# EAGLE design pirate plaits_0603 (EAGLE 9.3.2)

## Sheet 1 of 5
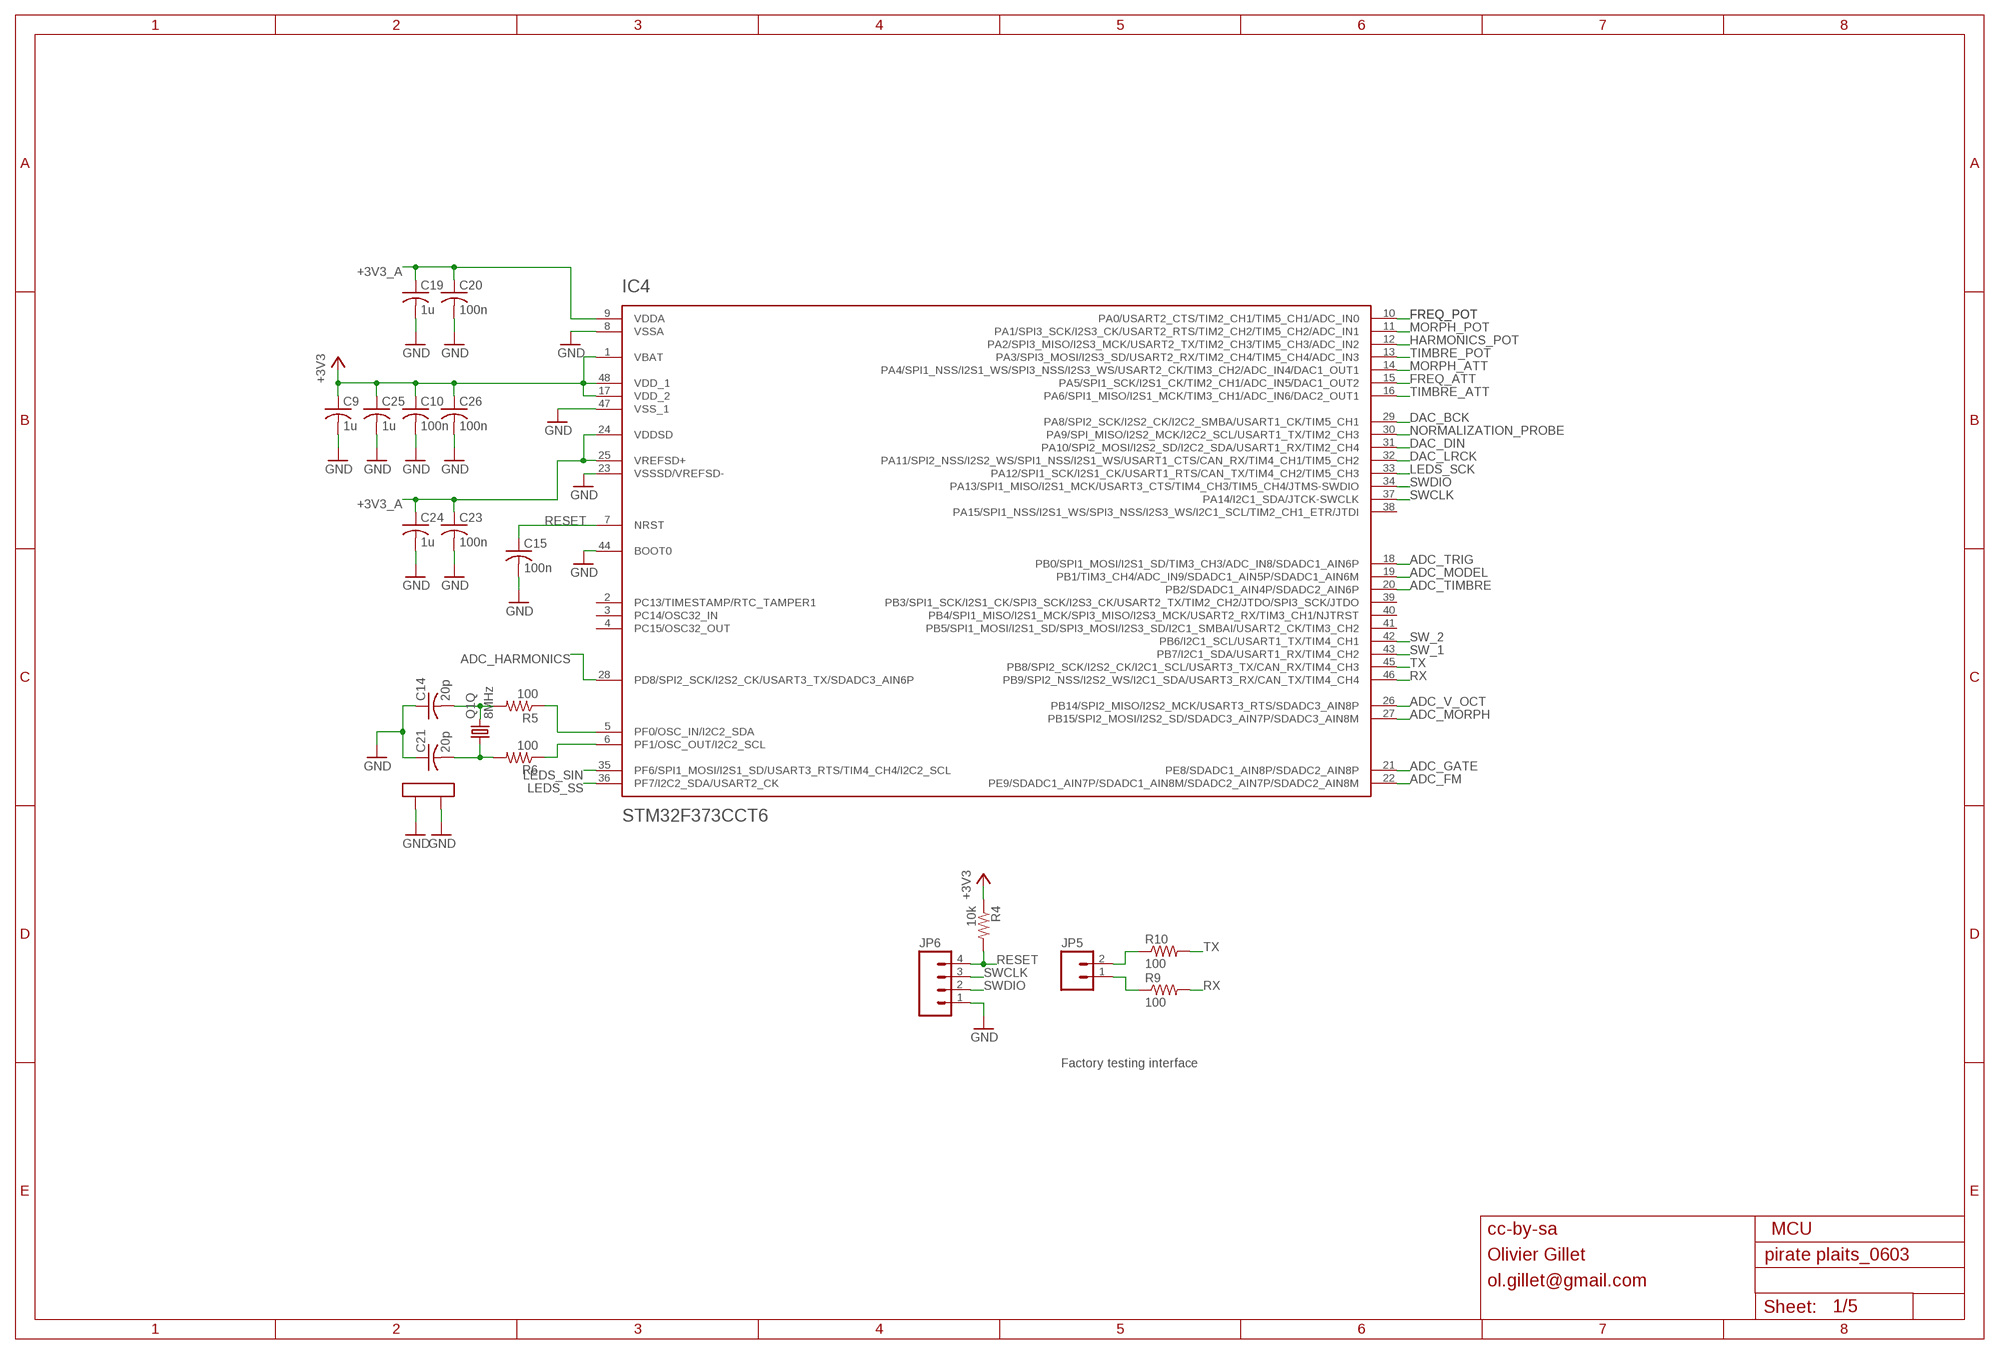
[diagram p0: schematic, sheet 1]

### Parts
C9  1u  C-USC0603  [C0603]
C10  100n  C-USC0603  [C0603]
C14  20p  C-USC0603  [C0603]
C15  100n  C-USC0603  [C0603]
C19  1u  C-USC0603  [C0603]
C20  100n  C-USC0603  [C0603]
C21  20p  C-USC0603  [C0603]
C23  100n  C-USC0603  [C0603]
C24  1u  C-USC0603  [C0603]
C25  1u  C-USC0603  [C0603]
C26  100n  C-USC0603  [C0603]
IC4  STM32F373CCT6  STM32F373C  [LQFP48]
JP5  M02PTH  [1X02]
JP6  M04PTH  [1X04]
Q1  8MHz  CRYSTAL  [CTS406]
R4  10k  R-US_R0603  [R0603]
R5  100  R-US_R0603  [R0603]
R6  100  R-US_R0603  [R0603]
R9  100  R-US_R0603  [R0603]
R10  100  R-US_R0603  [R0603]

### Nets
+3V3: C9.1 C10.1 C25.1 C26.1 IC4.1(VBAT) IC4.17(VDD_2) IC4.48(VDD_1) R4.1 ; also sheet 2,3,4,5
+3V3_A: C19.1 C20.1 C23.1 C24.1 IC4.9(VDDA) IC4.24(VDDSD) IC4.25(VREFSD+) ; also sheet 2,3,4,5
ADC_FM: IC4.22(PE9/SDADC1_AIN7P/SDADC1_AIN8M/SDADC2_AIN7P/SDADC2_AIN8M) ; also sheet 3
ADC_GATE: IC4.21(PE8/SDADC1_AIN8P/SDADC2_AIN8P) ; also sheet 3
ADC_HARMONICS: IC4.28(PD8/SPI2_SCK/I2S2_CK/USART3_TX/SDADC3_AIN6P) ; also sheet 3
ADC_MODEL: IC4.19(PB1/TIM3_CH4/ADC_IN9/SDADC1_AIN5P/SDADC1_AIN6M) ; also sheet 3
ADC_MORPH: IC4.27(PB15/SPI2_MOSI/I2S2_SD/SDADC3_AIN7P/SDADC3_AIN8M) ; also sheet 3
ADC_TIMBRE: IC4.20(PB2/SDADC1_AIN4P/SDADC2_AIN6P) ; also sheet 3
ADC_TRIG: IC4.18(PB0/SPI1_MOSI/I2S1_SD/TIM3_CH3/ADC_IN8/SDADC1_AIN6P) ; also sheet 3
ADC_V_OCT: IC4.26(PB14/SPI2_MISO/I2S2_MCK/USART3_RTS/SDADC3_AIN8P) ; also sheet 3
DAC_BCK: IC4.29(PA8/SPI2_SCK/I2S2_CK/I2C2_SMBA/USART1_CK/TIM5_CH1) ; also sheet 4
DAC_DIN: IC4.31(PA10/SPI2_MOSI/I2S2_SD/I2C2_SDA/USART1_RX/TIM2_CH4) ; also sheet 4
DAC_LRCK: IC4.32(PA11/SPI2_NSS/I2S2_WS/SPI1_NSS/I2S1_WS/USART1_CTS/CAN_RX/TIM4_CH1/TIM5_CH2) ; also sheet 4
FREQ_ATT: IC4.15(PA5/SPI1_SCK/I2S1_CK/TIM2_CH1/ADC_IN5/DAC1_OUT2) ; also sheet 2
FREQ_POT: IC4.10(PA0/USART2_CTS/TIM2_CH1/TIM5_CH1/ADC_IN0) ; also sheet 2
GND: C9.2 C10.2 C14.1 C15.2 C19.2 C20.2 C21.1 C23.2 C24.2 C25.2 C26.2 IC4.8(VSSA) IC4.23(VSSSD/VREFSD-) IC4.44(BOOT0) IC4.47(VSS_1) JP6.1 Q1.2(LID1) Q1.4(LID2) ; also sheet 2,3,4,5
HARMONICS_POT: IC4.12(PA2/SPI3_MISO/I2S3_MCK/USART2_TX/TIM2_CH3/TIM5_CH3/ADC_IN2) ; also sheet 2
LEDS_SCK: IC4.33(PA12/SPI1_SCK/I2S1_CK/USART1_RTS/CAN_TX/TIM4_CH2/TIM5_CH3) ; also sheet 2
LEDS_SIN: IC4.35(PF6/SPI1_MOSI/I2S1_SD/USART3_RTS/TIM4_CH4/I2C2_SCL) ; also sheet 2
LEDS_SS: IC4.36(PF7/I2C2_SDA/USART2_CK) ; also sheet 2
MORPH_ATT: IC4.14(PA4/SPI1_NSS/I2S1_WS/SPI3_NSS/I2S3_WS/USART2_CK/TIM3_CH2/ADC_IN4/DAC1_OUT1) ; also sheet 2
MORPH_POT: IC4.11(PA1/SPI3_SCK/I2S3_CK/USART2_RTS/TIM2_CH2/TIM5_CH2/ADC_IN1) ; also sheet 2
N$7: IC4.5(PF0/OSC_IN/I2C2_SDA) R5.1
N$8: IC4.6(PF1/OSC_OUT/I2C2_SCL) R6.1
N$29: C14.2 Q1.3 R5.2
N$33: JP5.2 R10.1
N$35: C21.2 Q1.1 R6.2
N$51: JP5.1 R9.1
NORMALIZATION_PROBE: IC4.30(PA9/SPI_MISO/I2S2_MCK/I2C2_SCL/USART1_TX/TIM2_CH3) ; also sheet 3
RESET: C15.1 IC4.7(NRST) JP6.4 R4.2
RX: IC4.46(PB9/SPI2_NSS/I2S2_WS/I2C1_SDA/USART3_RX/CAN_TX/TIM4_CH4) R9.2
SW_1: IC4.43(PB7/I2C1_SDA/USART1_RX/TIM4_CH2) ; also sheet 2
SW_2: IC4.42(PB6/I2C1_SCL/USART1_TX/TIM4_CH1) ; also sheet 2
SWCLK: IC4.37(PA14/I2C1_SDA/JTCK-SWCLK) JP6.3
SWDIO: IC4.34(PA13/SPI1_MISO/I2S1_MCK/USART3_CTS/TIM4_CH3/TIM5_CH4/JTMS-SWDIO) JP6.2
TIMBRE_ATT: IC4.16(PA6/SPI1_MISO/I2S1_MCK/TIM3_CH1/ADC_IN6/DAC2_OUT1) ; also sheet 2
TIMBRE_POT: IC4.13(PA3/SPI3_MOSI/I2S3_SD/USART2_RX/TIM2_CH4/TIM5_CH4/ADC_IN3) ; also sheet 2
TX: IC4.45(PB8/SPI2_SCK/I2S2_CK/I2C1_SCL/USART3_TX/CAN_RX/TIM4_CH3) R10.2
Unconnected: IC4.2(PC13/TIMESTAMP/RTC_TAMPER1) IC4.3(PC14/OSC32_IN) IC4.4(PC15/OSC32_OUT) IC4.38(PA15/SPI1_NSS/I2S1_WS/SPI3_NSS/I2S3_WS/I2C1_SCL/TIM2_CH1_ETR/JTDI) IC4.39(PB3/SPI1_SCK/I2S1_CK/SPI3_SCK/I2S3_CK/USART2_TX/TIM2_CH2/JTDO/SPI3_SCK/JTDO) IC4.40(PB4/SPI1_MISO/I2S1_MCK/SPI3_MISO/I2S3_MCK/USART2_RX/TIM3_CH1/NJTRST) IC4.41(PB5/SPI1_MOSI/I2S1_SD/SPI3_MOSI/I2S3_SD/I2C1_SMBAI/USART2_CK/TIM3_CH2)

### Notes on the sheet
- Factory testing interface
- cc-by-sa | MCU
- Olivier Gillet
- ol.gillet@gmail.com

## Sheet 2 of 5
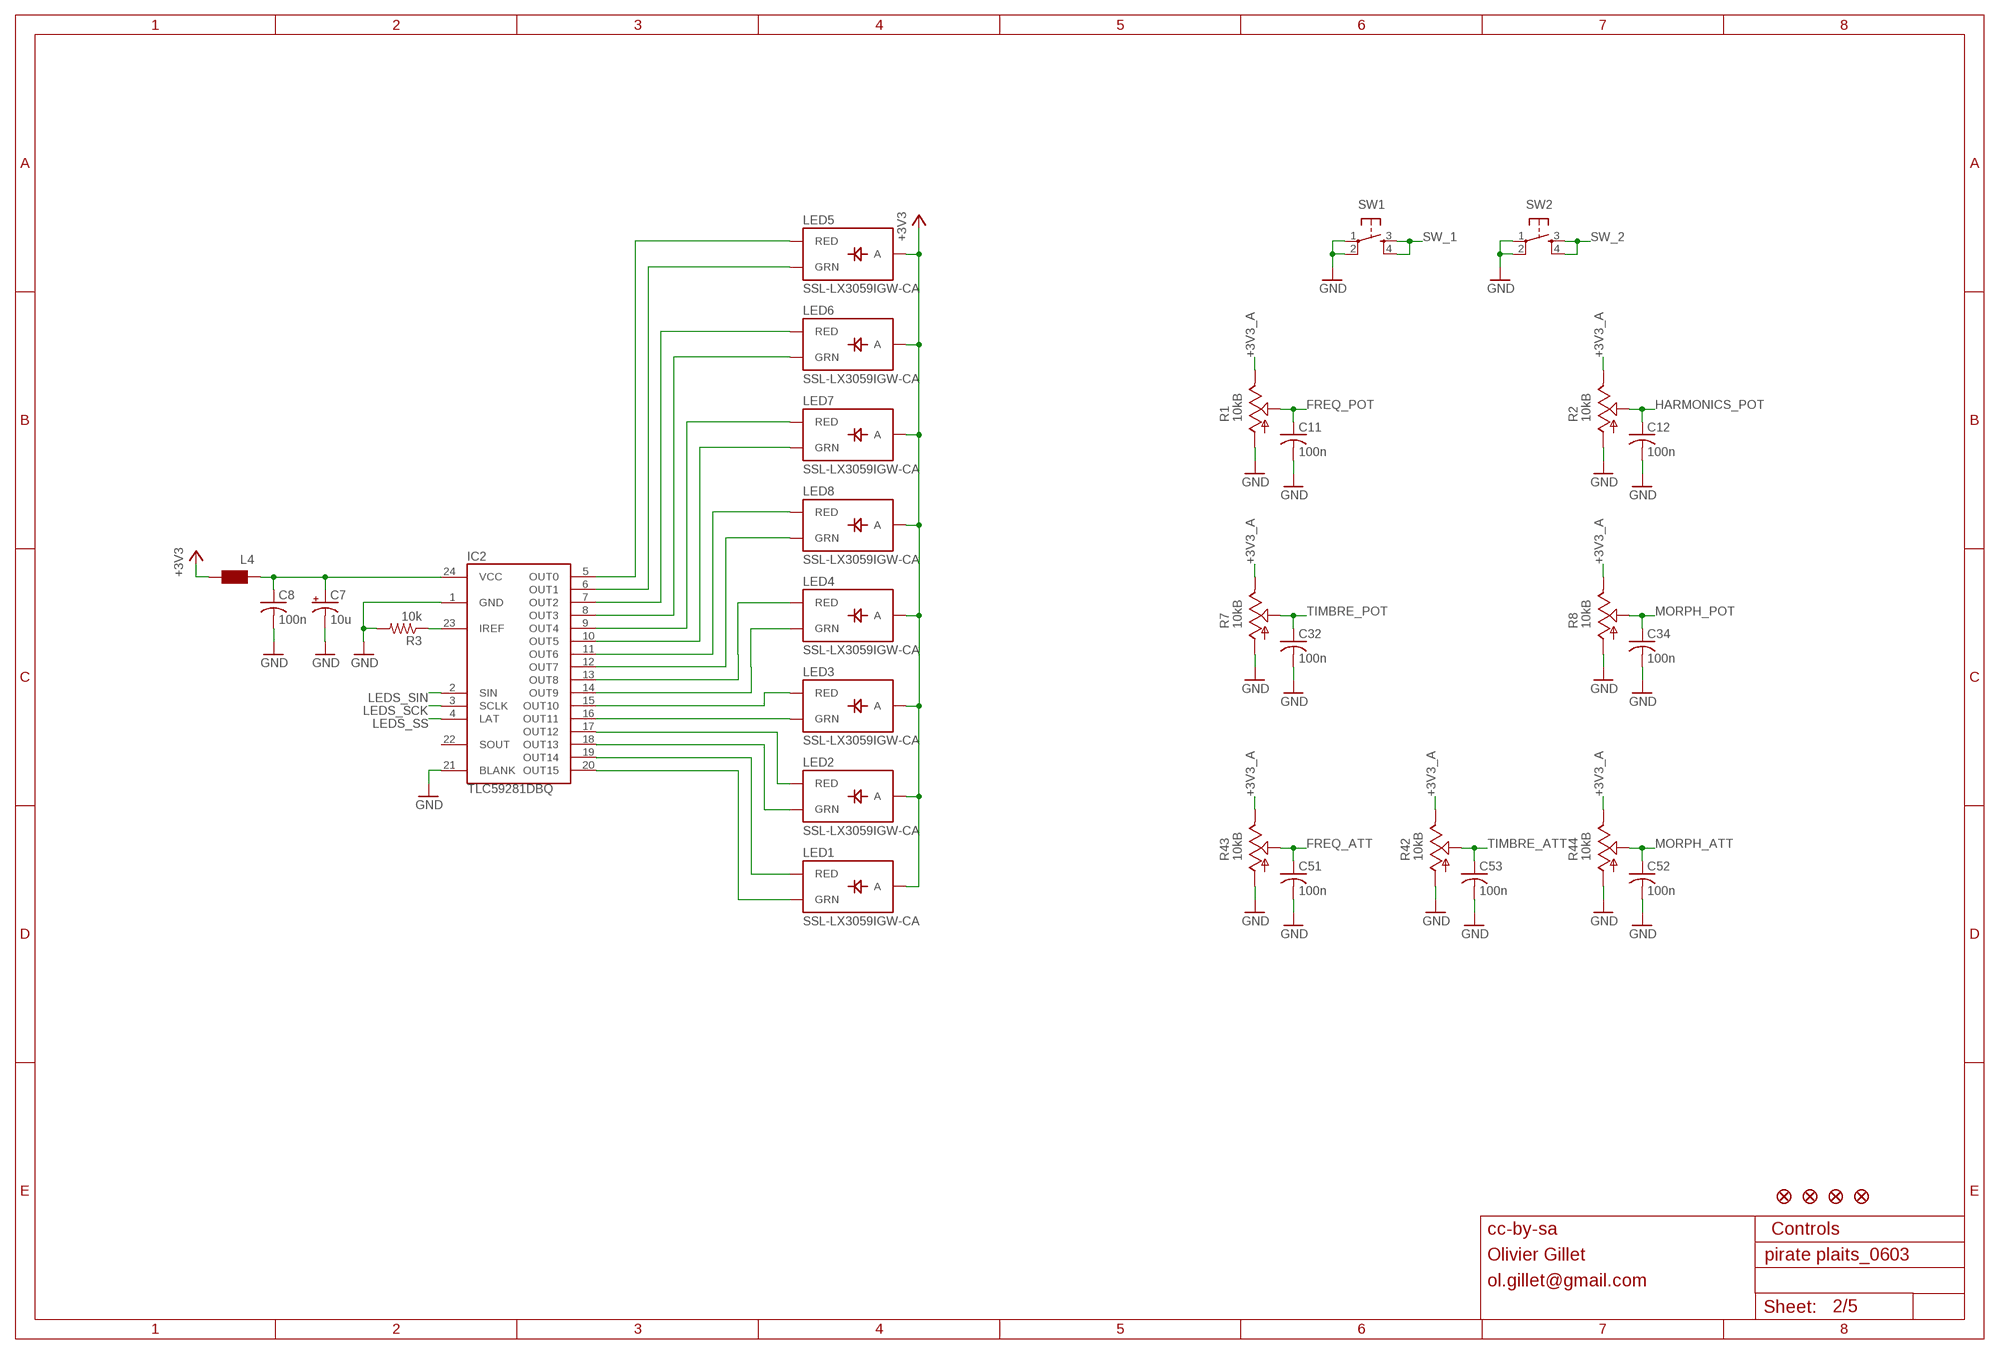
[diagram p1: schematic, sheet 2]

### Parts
C7  10u  CPOL-USA  [PANASONIC_A]
C8  100n  C-USC0603  [C0603]
C11  100n  C-USC0603  [C0603]
C12  100n  C-USC0603  [C0603]
C32  100n  C-USC0603  [C0603]
C34  100n  C-USC0603  [C0603]
C51  100n  C-USC0603  [C0603]
C52  100n  C-USC0603  [C0603]
C53  100n  C-USC0603  [C0603]
IC2  TLC59281DBQ  [TSSOP24_0635]
JP1  FIDUCIAL1X2  [FIDUCIAL-1X2]
JP2  FIDUCIAL1X2  [FIDUCIAL-1X2]
JP3  FIDUCIAL1X2  [FIDUCIAL-1X2]
JP4  FIDUCIAL1X2  [FIDUCIAL-1X2]
L4  WE-CBF_0603  [0603]
LED1  SSL-LX3059IGW-CA  LED-BICOLOR-THROUGHHOLE-CA  [LED-BICOLOR-THROUGHHOLE-LUMEX]
LED2  SSL-LX3059IGW-CA  LED-BICOLOR-THROUGHHOLE-CA  [LED-BICOLOR-THROUGHHOLE-LUMEX]
LED3  SSL-LX3059IGW-CA  LED-BICOLOR-THROUGHHOLE-CA  [LED-BICOLOR-THROUGHHOLE-LUMEX]
LED4  SSL-LX3059IGW-CA  LED-BICOLOR-THROUGHHOLE-CA  [LED-BICOLOR-THROUGHHOLE-LUMEX]
LED5  SSL-LX3059IGW-CA  LED-BICOLOR-THROUGHHOLE-CA  [LED-BICOLOR-THROUGHHOLE-LUMEX]
LED6  SSL-LX3059IGW-CA  LED-BICOLOR-THROUGHHOLE-CA  [LED-BICOLOR-THROUGHHOLE-LUMEX]
LED7  SSL-LX3059IGW-CA  LED-BICOLOR-THROUGHHOLE-CA  [LED-BICOLOR-THROUGHHOLE-LUMEX]
LED8  SSL-LX3059IGW-CA  LED-BICOLOR-THROUGHHOLE-CA  [LED-BICOLOR-THROUGHHOLE-LUMEX]
R1  10kB  POT_USVERTICAL_PS  [ALPS_POT_VERTICAL_PS]
R2  10kB  POT_USVERTICAL_PS  [ALPS_POT_VERTICAL_PS]
R3  10k  R-US_R0603  [R0603]
R7  10kB  POT_USVERTICAL_PS  [ALPS_POT_VERTICAL_PS]
R8  10kB  POT_USVERTICAL_PS  [ALPS_POT_VERTICAL_PS]
R42  10kB  POT_USVERTICAL  [ALPS_POT_VERTICAL]
R43  10kB  POT_USVERTICAL  [ALPS_POT_VERTICAL]
R44  10kB  POT_USVERTICAL  [ALPS_POT_VERTICAL]
SW1  TAC_SWITCHPTH  [TACTILE-PTH]
SW2  TAC_SWITCHPTH  [TACTILE-PTH]

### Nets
+3V3: L4.2 LED1.A LED2.A LED3.A LED4.A LED5.A LED6.A LED7.A LED8.A ; also sheet 1,3,4,5
+3V3_A: R1.P$1(E) R2.P$1(E) R7.P$1(E) R8.P$1(E) R42.P$1(E) R43.P$1(E) R44.P$1(E) ; also sheet 1,3,4,5
FREQ_ATT: C51.1 R43.P$2(S) ; also sheet 1
FREQ_POT: C11.1 R1.P$2(S) ; also sheet 1
GND: C7.- C8.2 C11.2 C12.2 C32.2 C34.2 C51.2 C52.2 C53.2 IC2.1(GND) IC2.21(BLANK) R1.P$3(A) R2.P$3(A) R3.2 R7.P$3(A) R8.P$3(A) R42.P$3(A) R43.P$3(A) R44.P$3(A) SW1.1 SW1.2 SW2.1 SW2.2 ; also sheet 1,3,4,5
HARMONICS_POT: C12.1 R2.P$2(S) ; also sheet 1
LEDS_SCK: IC2.3(SCLK) ; also sheet 1
LEDS_SIN: IC2.2(SIN) ; also sheet 1
LEDS_SS: IC2.4(LAT) ; also sheet 1
MORPH_ATT: C52.1 R44.P$2(S) ; also sheet 1
MORPH_POT: C34.1 R8.P$2(S) ; also sheet 1
N$2: IC2.12(OUT7) LED8.GREEN_C(GRN)
N$5: IC2.11(OUT6) LED8.RED_C(RED)
N$9: IC2.10(OUT5) LED7.GREEN_C(GRN)
N$10: IC2.9(OUT4) LED7.RED_C(RED)
N$11: IC2.8(OUT3) LED6.GREEN_C(GRN)
N$12: IC2.13(OUT8) LED4.RED_C(RED)
N$13: IC2.7(OUT2) LED6.RED_C(RED)
N$14: IC2.14(OUT9) LED4.GREEN_C(GRN)
N$15: IC2.6(OUT1) LED5.GREEN_C(GRN)
N$17: IC2.15(OUT10) LED3.RED_C(RED)
N$18: IC2.16(OUT11) LED3.GREEN_C(GRN)
N$19: IC2.17(OUT12) LED2.RED_C(RED)
N$20: IC2.18(OUT13) LED2.GREEN_C(GRN)
N$21: IC2.19(OUT14) LED1.RED_C(RED)
N$22: IC2.5(OUT0) LED5.RED_C(RED)
N$23: IC2.20(OUT15) LED1.GREEN_C(GRN)
N$27: C7.+ C8.1 IC2.24(VCC) L4.1
N$68: IC2.23(IREF) R3.1
SW_1: SW1.3 SW1.4 ; also sheet 1
SW_2: SW2.3 SW2.4 ; also sheet 1
TIMBRE_ATT: C53.1 R42.P$2(S) ; also sheet 1
TIMBRE_POT: C32.1 R7.P$2(S) ; also sheet 1
Unconnected: IC2.22(SOUT)

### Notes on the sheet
- cc-by-sa | Controls
- Olivier Gillet
- ol.gillet@gmail.com

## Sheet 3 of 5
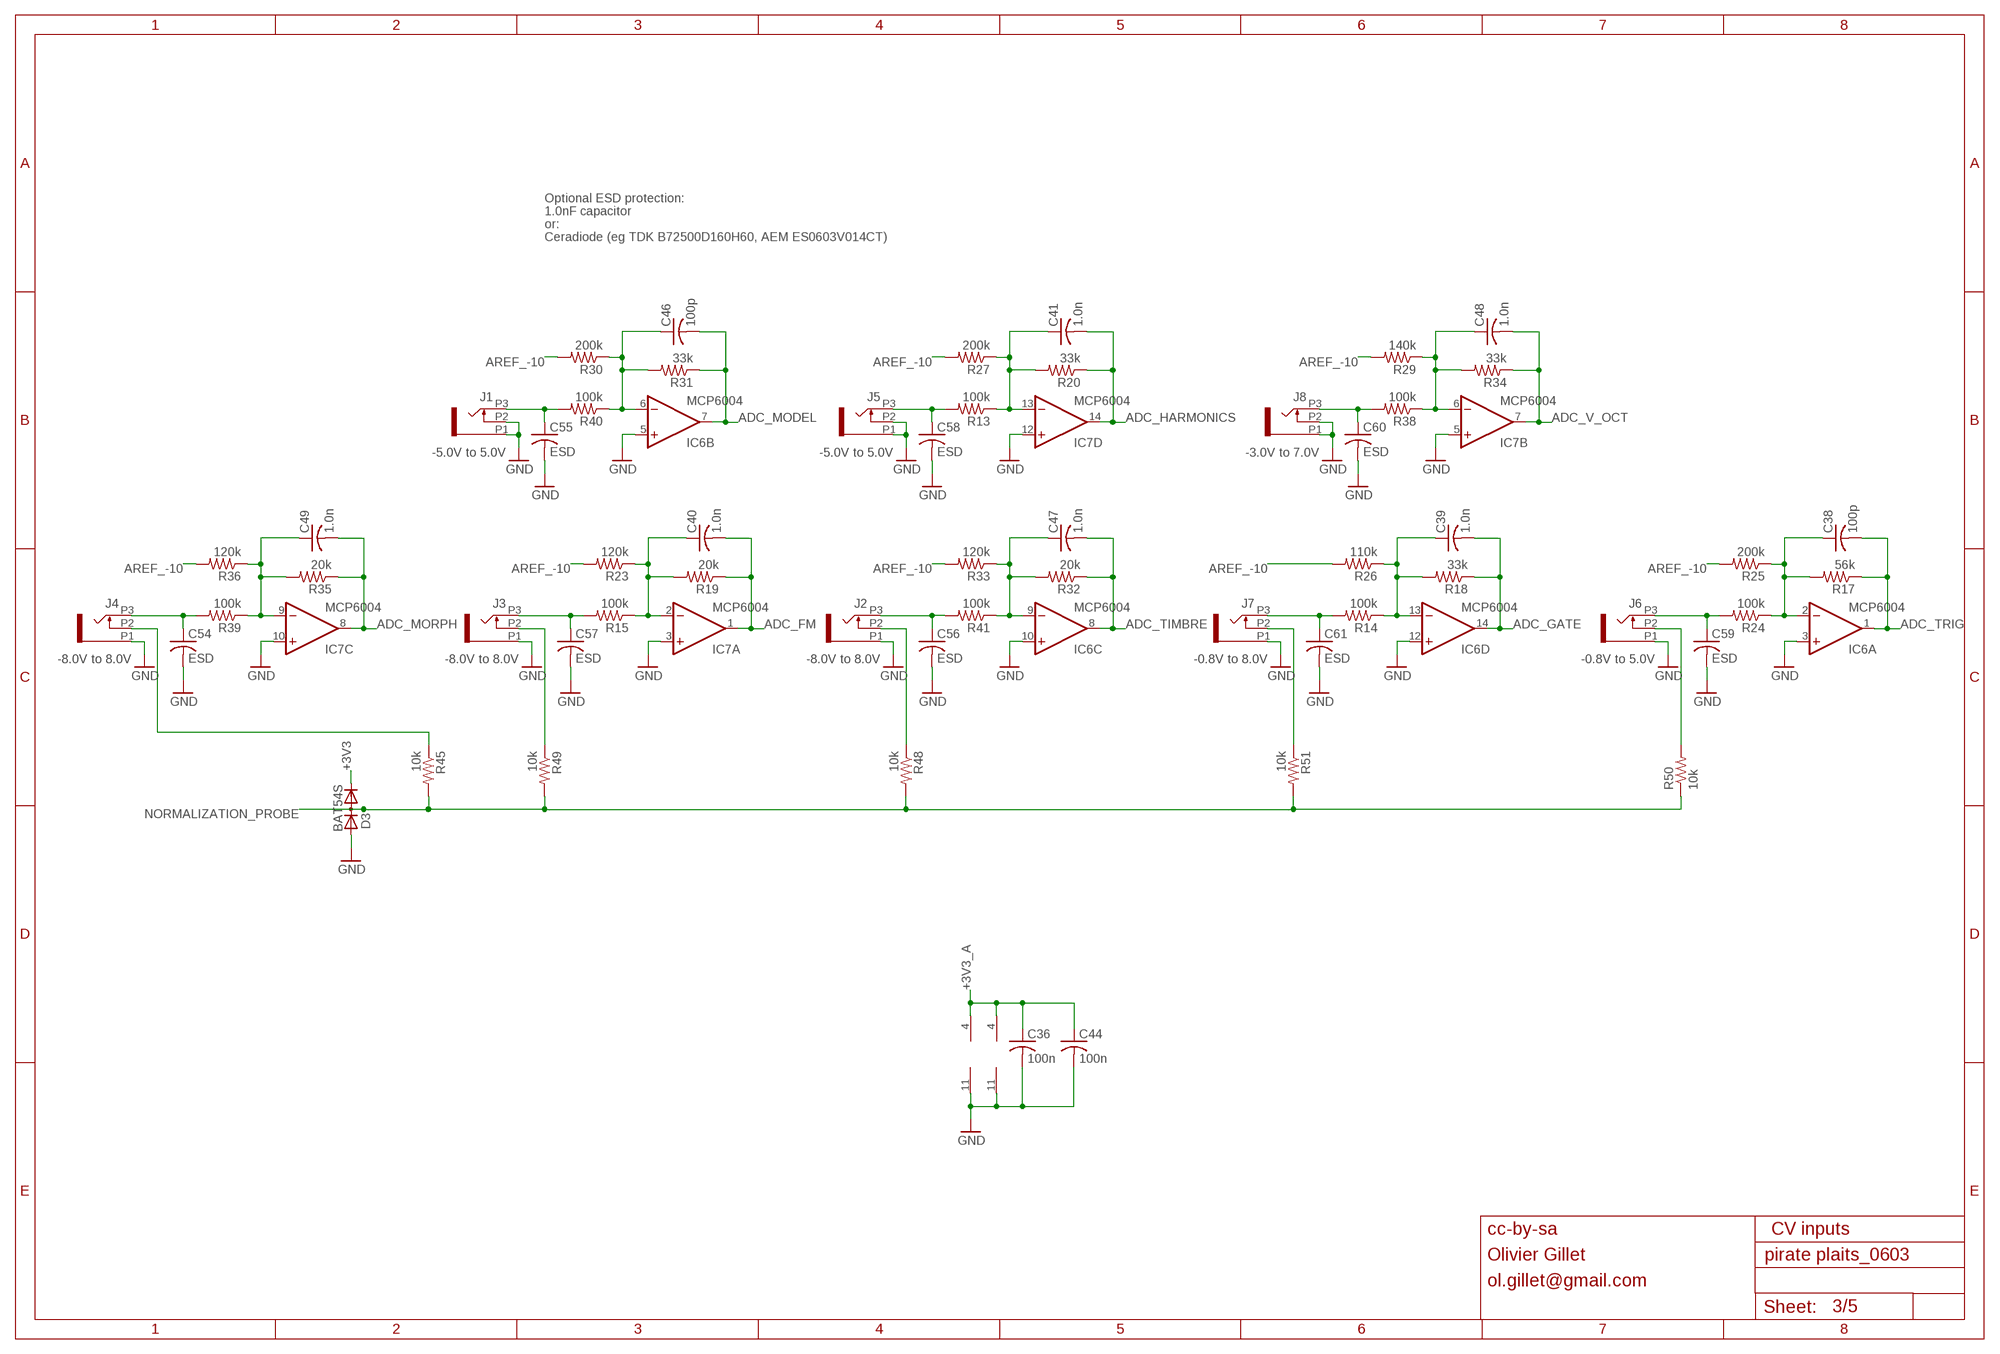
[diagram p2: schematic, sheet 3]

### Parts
C36  100n  C-USC0603  [C0603]
C38  100p  C-USC0603  [C0603]
C39  1.0n  C-USC0603  [C0603]
C40  1.0n  C-USC0603  [C0603]
C41  1.0n  C-USC0603  [C0603]
C44  100n  C-USC0603  [C0603]
C46  100p  C-USC0603  [C0603]
C47  1.0n  C-USC0603  [C0603]
C48  1.0n  C-USC0603  [C0603]
C49  1.0n  C-USC0603  [C0603]
C54  ESD  C-USC0603  [C0603]
C55  ESD  C-USC0603  [C0603]
C56  ESD  C-USC0603  [C0603]
C57  ESD  C-USC0603  [C0603]
C58  ESD  C-USC0603  [C0603]
C59  ESD  C-USC0603  [C0603]
C60  ESD  C-USC0603  [C0603]
C61  ESD  C-USC0603  [C0603]
D3  BAT54S  DIODE_2CACA-SOT23  [SOT23]
IC6  MCP6004  TL074PW  [TSSOP14_065]
IC7  MCP6004  TL074PW  [TSSOP14_065]
J1  PJ301_THONKICONN6  [WQP_PJ_301M6]
J2  PJ301_THONKICONN6  [WQP_PJ_301M6]
J3  PJ301_THONKICONN6  [WQP_PJ_301M6]
J4  PJ301_THONKICONN6  [WQP_PJ_301M6]
J5  PJ301_THONKICONN6  [WQP_PJ_301M6]
J6  PJ301_THONKICONN6  [WQP_PJ_301M6]
J7  PJ301_THONKICONN6  [WQP_PJ_301M6]
J8  PJ301_THONKICONN6  [WQP_PJ_301M6]
R13  100k  R-US_R0603  [R0603]
R14  100k  R-US_R0603  [R0603]
R15  100k  R-US_R0603  [R0603]
R17  56k  R-US_R0603  [R0603]
R18  33k  R-US_R0603  [R0603]
R19  20k  R-US_R0603  [R0603]
R20  33k  R-US_R0603  [R0603]
R23  120k  R-US_R0603  [R0603]
R24  100k  R-US_R0603  [R0603]
R25  200k  R-US_R0603  [R0603]
R26  110k  R-US_R0603  [R0603]
R27  200k  R-US_R0603  [R0603]
R29  140k  R-US_R0603  [R0603]
R30  200k  R-US_R0603  [R0603]
R31  33k  R-US_R0603  [R0603]
R32  20k  R-US_R0603  [R0603]
R33  120k  R-US_R0603  [R0603]
R34  33k  R-US_R0603  [R0603]
R35  20k  R-US_R0603  [R0603]
R36  120k  R-US_R0603  [R0603]
R38  100k  R-US_R0603  [R0603]
R39  100k  R-US_R0603  [R0603]
R40  100k  R-US_R0603  [R0603]
R41  100k  R-US_R0603  [R0603]
R45  10k  R-US_R0603  [R0603]
R48  10k  R-US_R0603  [R0603]
R49  10k  R-US_R0603  [R0603]
R50  10k  R-US_R0603  [R0603]
R51  10k  R-US_R0603  [R0603]

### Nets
+3V3: D3.2(C) ; also sheet 1,2,4,5
+3V3_A: C36.1 C44.1 IC6.4(P:V+) IC7.4(P:V+) ; also sheet 1,2,4,5
ADC_FM: C40.2 IC7.1(A:OUT) R19.1 ; also sheet 1
ADC_GATE: C39.2 IC6.14(D:OUT) R18.1 ; also sheet 1
ADC_HARMONICS: C41.2 IC7.14(D:OUT) R20.1 ; also sheet 1
ADC_MODEL: C46.2 IC6.7(B:OUT) R31.1 ; also sheet 1
ADC_MORPH: C49.2 IC7.8(C:OUT) R35.1 ; also sheet 1
ADC_TIMBRE: C47.2 IC6.8(C:OUT) R32.1 ; also sheet 1
ADC_TRIG: C38.2 IC6.1(A:OUT) R17.1 ; also sheet 1
ADC_V_OCT: C48.2 IC7.7(B:OUT) R34.1 ; also sheet 1
AREF_-10: R23.2 R25.2 R26.2 R27.2 R29.2 R30.2 R33.2 R36.2 ; also sheet 5
FM_IN: C57.1 J3.P3 R15.2
GATE_IN: C61.1 J7.P3 R14.2
GATE_IN1: C59.1 J6.P3 R24.2
GND: C36.2 C44.2 C54.2 C55.2 C56.2 C57.2 C58.2 C59.2 C60.2 C61.2 D3.1(A) IC6.3(A:+IN) IC6.5(B:+IN) IC6.10(C:+IN) IC6.11(P:V-) IC6.12(D:+IN) IC7.3(A:+IN) IC7.5(B:+IN) IC7.10(C:+IN) IC7.11(P:V-) IC7.12(D:+IN) J1.P1 J1.P2 J2.P1 J3.P1 J4.P1 J5.P1 J5.P2 J6.P1 J7.P1 J8.P1 J8.P2 ; also sheet 1,2,4,5
HARMONICS_IN: C58.1 J5.P3 R13.2
MODEL_IN: C55.1 J1.P3 R40.2
MORPH_IN: C54.1 J4.P3 R39.2
N$3: J6.P2 R50.2
N$4: C38.1 IC6.2(A:-IN) R17.2 R24.1 R25.1
N$24: J3.P2 R49.1
N$25: J2.P2 R48.1
N$26: J4.P2 R45.1
N$28: C39.1 IC6.13(D:-IN) R14.1 R18.2 R26.1
N$30: C48.1 IC7.6(B:-IN) R29.1 R34.2 R38.1
N$31: C56.1 J2.P3 R41.2
N$32: C49.1 IC7.9(C:-IN) R35.2 R36.1 R39.1
N$34: C40.1 IC7.2(A:-IN) R15.1 R19.2 R23.1
N$36: J7.P2 R51.1
N$37: C46.1 IC6.6(B:-IN) R30.1 R31.2 R40.1
N$39: C47.1 IC6.9(C:-IN) R32.2 R33.1 R41.1
N$41: C41.1 IC7.13(D:-IN) R13.1 R20.2 R27.1
NORMALIZATION_PROBE: D3.3(AC) R45.2 R48.2 R49.2 R50.1 R51.2 ; also sheet 1
V_OCT_IN: C60.1 J8.P3 R38.2

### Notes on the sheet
- Optional ESD protection:
- 1.0nF capacitor
- or:
- Ceradiode (eg TDK B72500D160H60, AEM ES0603V014CT)
- -5.0V to 5.0V | -5.0V to 5.0V | -3.0V to 7.0V
- -8.0V to 8.0V | -8.0V to 8.0V | -8.0V to 8.0V | -0.8V to 8.0V | -0.8V to 5.0V
- cc-by-sa | CV inputs
- Olivier Gillet
- ol.gillet@gmail.com

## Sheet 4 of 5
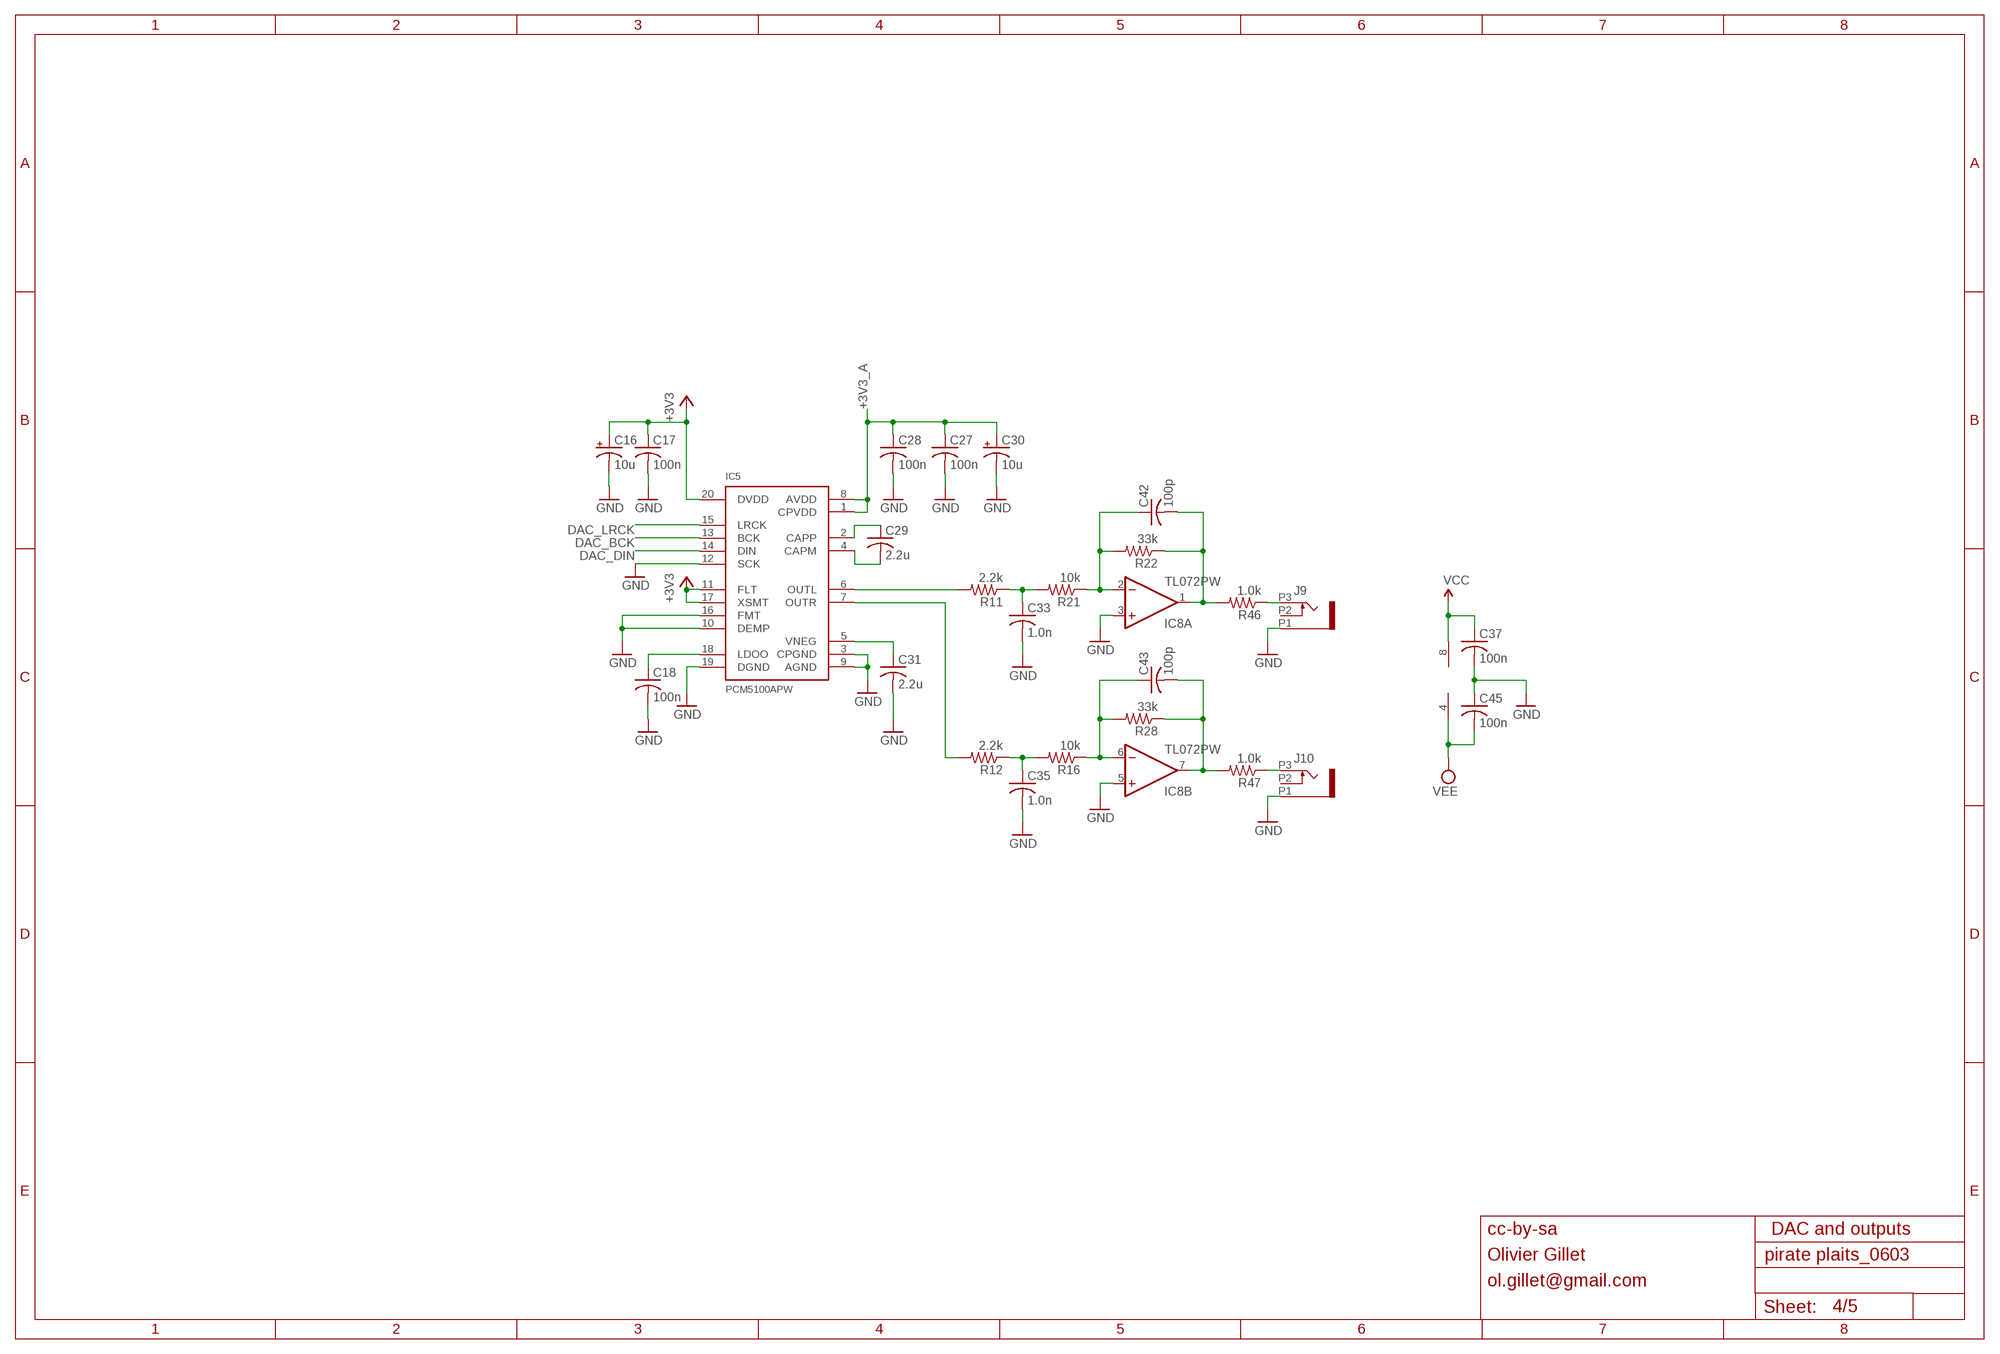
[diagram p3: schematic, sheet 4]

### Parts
C16  10u  CPOL-USA  [PANASONIC_A]
C17  100n  C-USC0603  [C0603]
C18  100n  C-USC0603  [C0603]
C27  100n  C-USC0603  [C0603]
C28  100n  C-USC0603  [C0603]
C29  2.2u  C-USC0805  [C0805]
C30  10u  CPOL-USA  [PANASONIC_A]
C31  2.2u  C-USC0805  [C0805]
C33  1.0n  C-USC0603  [C0603]
C35  1.0n  C-USC0603  [C0603]
C37  100n  C-USC0603  [C0603]
C42  100p  C-USC0603  [C0603]
C43  100p  C-USC0603  [C0603]
C45  100n  C-USC0603  [C0603]
IC5  PCM5100APW  PCM5100PW  [SSOP20]
IC8  TL072PW  [TSSOP08]
J9  PJ301_THONKICONN6  [WQP_PJ_301M6]
J10  PJ301_THONKICONN6  [WQP_PJ_301M6]
R11  2.2k  R-US_R0603  [R0603]
R12  2.2k  R-US_R0603  [R0603]
R16  10k  R-US_R0603  [R0603]
R21  10k  R-US_R0603  [R0603]
R22  33k  R-US_R0603  [R0603]
R28  33k  R-US_R0603  [R0603]
R46  1.0k  R-US_R0603  [R0603]
R47  1.0k  R-US_R0603  [R0603]

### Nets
+3V3: C16.+ C17.1 IC5.11(FLT) IC5.17(XSMT) IC5.20(DVDD) ; also sheet 1,2,3,5
+3V3_A: C27.1 C28.1 C30.+ IC5.1(CPVDD) IC5.8(AVDD) ; also sheet 1,2,3,5
DAC_BCK: IC5.13(BCK) ; also sheet 1
DAC_DIN: IC5.14(DIN) ; also sheet 1
DAC_LRCK: IC5.15(LRCK) ; also sheet 1
GND: C16.- C17.2 C18.2 C27.2 C28.2 C30.- C31.2 C33.2 C35.2 C37.2 C45.1 IC5.3(CPGND) IC5.9(AGND) IC5.10(DEMP) IC5.12(SCK) IC5.16(FMT) IC5.19(DGND) IC8.3(A:+IN) IC8.5(B:+IN) J9.P1 J10.P1 ; also sheet 1,2,3,5
N$6: C29.1 IC5.2(CAPP)
N$16: C29.2 IC5.4(CAPM)
N$43: IC5.6(OUTL) R11.2
N$46: C33.1 R11.1 R21.2
N$47: C35.1 R12.1 R16.2
N$48: C31.1 IC5.5(VNEG)
N$54: C18.1 IC5.18(LDOO)
N$55: IC5.7(OUTR) R12.2
N$58: C43.1 IC8.6(B:-IN) R16.1 R28.2
N$60: C43.2 IC8.7(B:OUT) R28.1 R47.2
N$62: C42.1 IC8.2(A:-IN) R21.1 R22.2
N$63: C42.2 IC8.1(A:OUT) R22.1 R46.2
N$65: J9.P3 R46.1
N$69: J10.P3 R47.1
VCC: C37.1 IC8.8(P:V+) ; also sheet 5
VEE: C45.2 IC8.4(P:V-) ; also sheet 5
Unconnected: J9.P2 J10.P2

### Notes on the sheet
- cc-by-sa | DAC and outputs
- Olivier Gillet
- ol.gillet@gmail.com

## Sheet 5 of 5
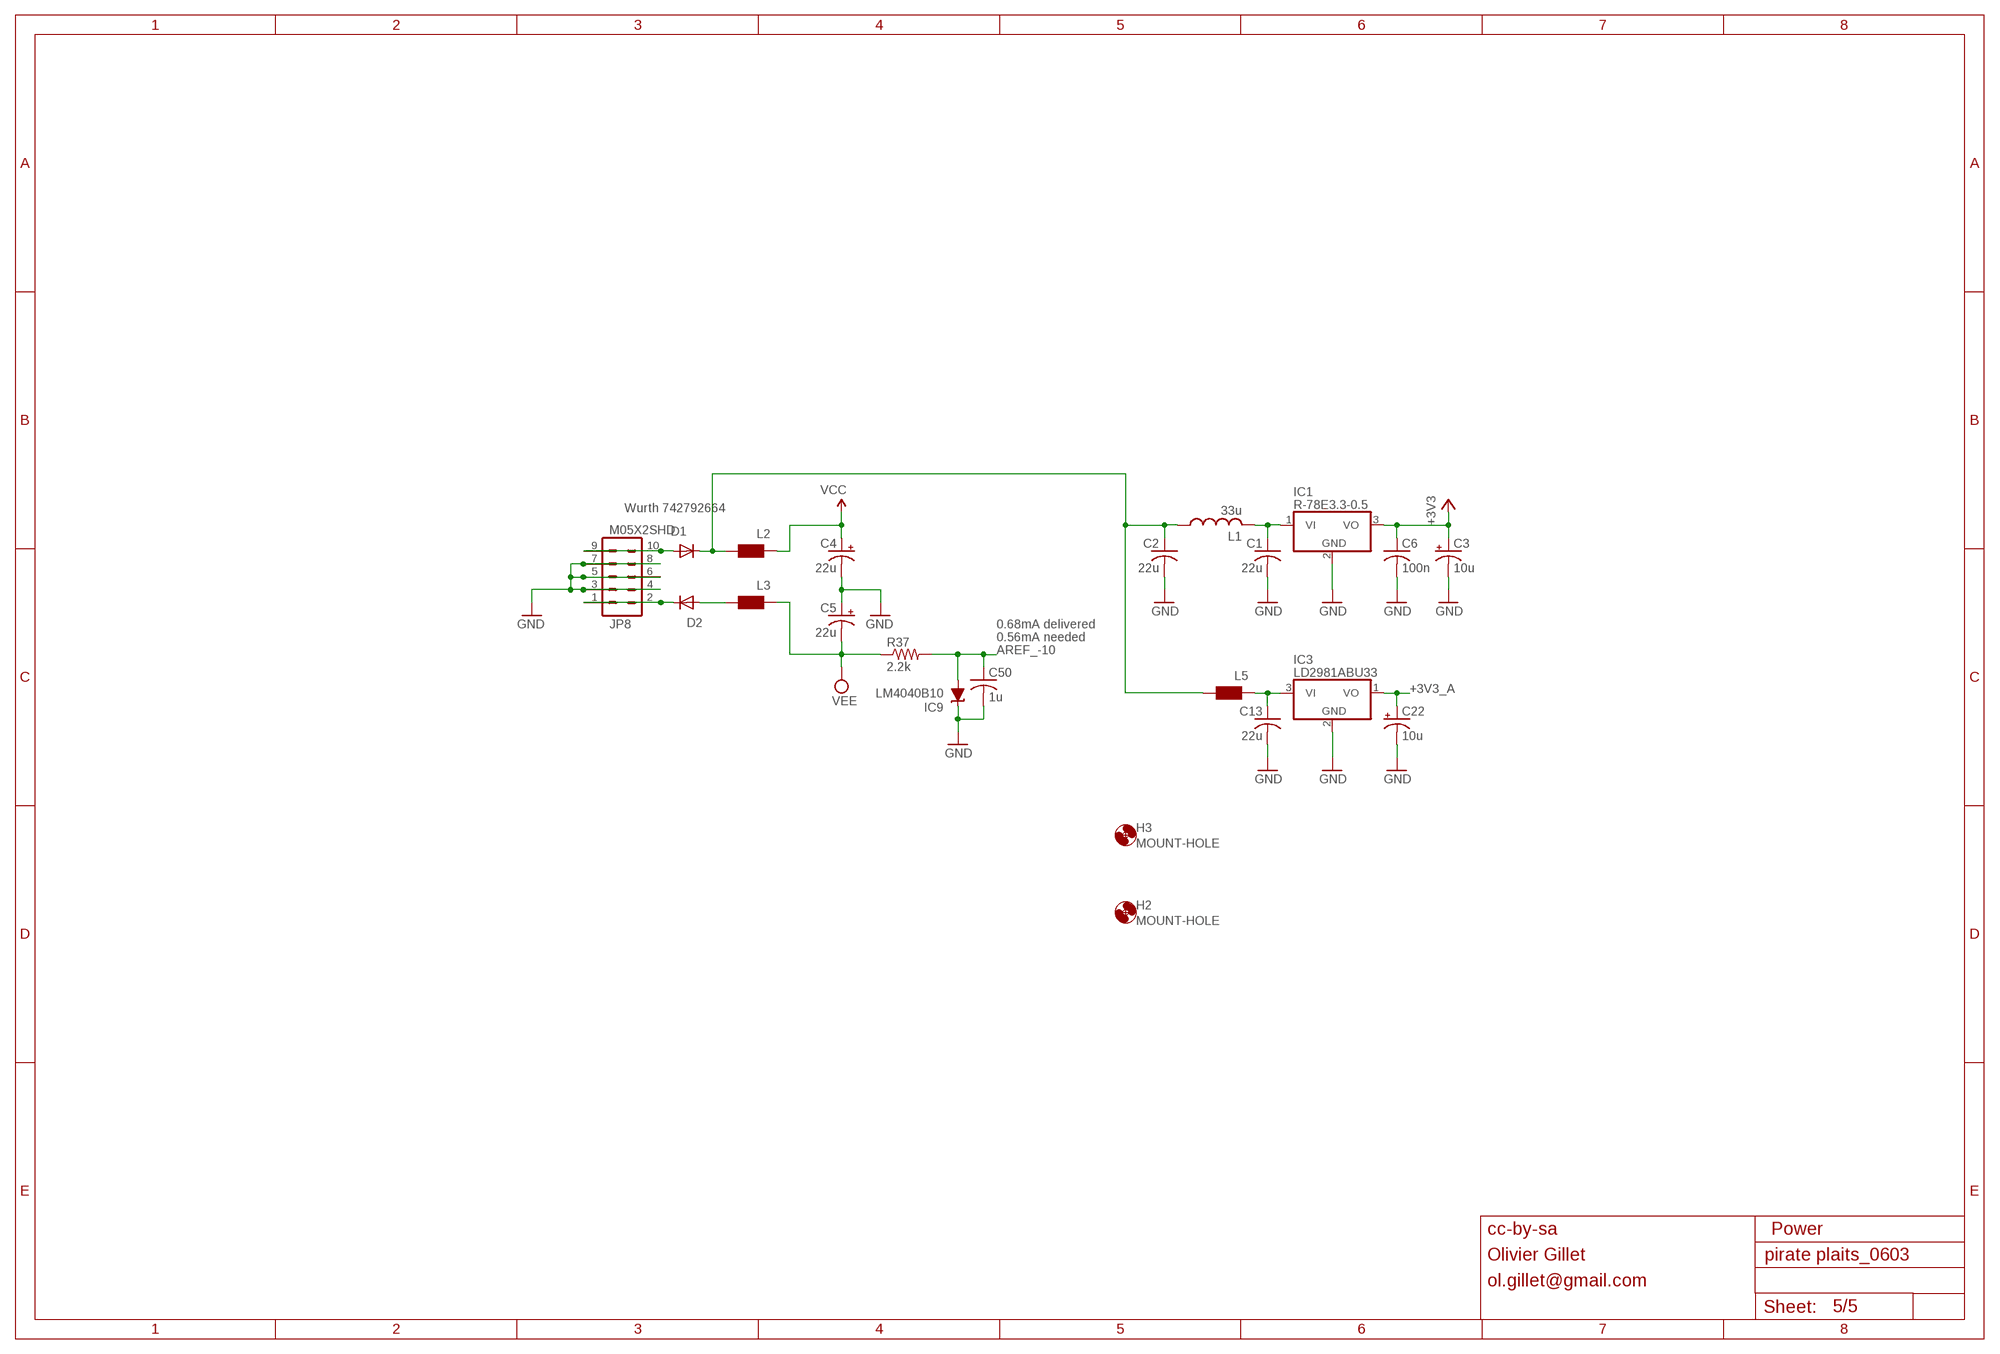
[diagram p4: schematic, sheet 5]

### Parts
C1  22u  C-USC1206  [C1206]
C2  22u  C-USC1206  [C1206]
C3  10u  CPOL-USA  [PANASONIC_A]
C4  22u  CPOL-USB  [PANASONIC_B]
C5  22u  CPOL-USB  [PANASONIC_B]
C6  100n  C-USC0603  [C0603]
C13  22u  C-USC1206  [C1206]
C22  10u  CPOL-USA  [PANASONIC_A]
C50  1u  C-USC0603  [C0603]
D1  1N5819HW  DIODE-SOD123  [SOD123]
D2  1N5819HW  DIODE-SOD123  [SOD123]
H2  MOUNT-HOLE  MOUNT-HOLE3.0TINY  [3,0TINY]
H3  MOUNT-HOLE  MOUNT-HOLE3.0TINY  [3,0TINY]
IC1  R-78E3.3-0.5  WE173950378  [WE78]
IC3  LD2981ABU33  LD2981ABU  [SOT89]
IC9  LM4040B10  LM4041B12DBZ  [DBZ_R-PDSO-G3]
JP8  M05X2SHD  [2X5-SHROUDED]
L1  33u  L-USL2012C  [L2012C]
L2  WE-CBF_0603  [0603]
L3  WE-CBF_0603  [0603]
L5  WE-CBF_0603  [0603]
R37  2.2k  R-US_R0603  [R0603]

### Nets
+3V3: C3.+ C6.1 IC1.3(VO) ; also sheet 1,2,3,4
+3V3_A: C22.+ IC3.1(VO) ; also sheet 1,2,3,4
AREF_-10: C50.1 IC9.2(A) R37.2 ; also sheet 3
GND: C1.2 C2.2 C3.- C4.- C5.+ C6.2 C13.2 C22.- C50.2 IC1.2(GND) IC3.2(GND) IC9.1(C) JP8.3 JP8.4 JP8.5 JP8.6 JP8.7 JP8.8 ; also sheet 1,2,3,4
N$1: C1.1 IC1.1(VI) L1.2
N$38: D2.A L3.2
N$40: C2.1 D1.C L1.1 L2.2 L5.2
N$42: C13.1 IC3.3(VI) L5.1
N$56: D1.A JP8.9 JP8.10
N$64: D2.C JP8.1 JP8.2
VCC: C4.+ L2.1 ; also sheet 4
VEE: C5.- L3.1 R37.1 ; also sheet 4

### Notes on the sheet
- Wurth 742792664
- 0.68mA delivered
- 0.56mA needed
- cc-by-sa | Power
- Olivier Gillet
- ol.gillet@gmail.com

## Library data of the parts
C1 C2 C13 C29 C31 C54-C61 = rcl:C-US: CAPACITOR, American symbol
C3-C5 C7 C16 C22 C30 = rcl:CPOL-US: POLARIZED CAPACITOR, American symbol
C6 C8-C12 C14 C15 C17-C21 C23-C28 C32-C53 = resistor:C-US: CAPACITOR, American symbol
D1 D2 = diode:DIODE-: DIODE
D3 = diode:DIODE_2CACA-: 2 Diodes - Cathode-Anode|Cathode-Anode
H2 H3 = og-holes:MOUNT-HOLE: MOUNTING HOLE with drill center marker
IC1 = og-vreg:WE173950378
IC2 = og-ics:TLC59281
IC3 = og-vreg:LD2981
IC4 = og-stm32f2:STM32F373C
IC5 = og-dac:PCM5100
IC6 IC7 = og-linear:TL074: OP AMP
IC8 = og-linear:TL072: OP AMP
IC9 = texas:LM4041: PRECISION MICROPOWER SHUNT VOLTAGE REFERENCE
J1-J10 = og-pj301_variations:PJ301_THONKICONN
JP1-JP4 = SparkFun:FIDUCIAL: Fiducial Alignment Points
JP5 = SparkFun:M02: Header 2
JP6 = SparkFun:M04: Header 4 Standard 4-pin 0.1" header. Use with straight break away headers (SKU : PRT-00116), right angle break away headers (PRT-00553), swiss pins (PRT-00743), machine pins (PRT-00117), and female headers (PRT-00115). Molex polarized connector foot print use with SKU : PRT-08231 with associated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
JP8 = og-header:M05X2: Header 5x2 Standard 10-pin dual row 0.1" header. Commonly used with AVR-ISP. Use with Spark Fun Electronics SKU: PRT-00778
L1 = og-rcl:L-US
L2-L5 = wuerth-elektronik:WE-CBF: SMD EMI Suppression Ferrite Beads
LED1-LED8 = og-leds:LED-BICOLOR-THROUGHHOLE-CA
Q1 = og-crystal:CRYSTAL: Crystal with 2 extra terminals for the metal LID (Abracon ABMM2 for example)
R1 R2 R7 R8 R42-R44 = og-pots:POT_US
R3-R6 R9-R41 R45-R51 = resistor:R-US_: RESISTOR, American symbol
SW1 SW2 = SparkFun:TAC_SWITCH: Momentary Switch Button commonly used for reset or general input. Spark Fun Electronics SKU : COM-00097

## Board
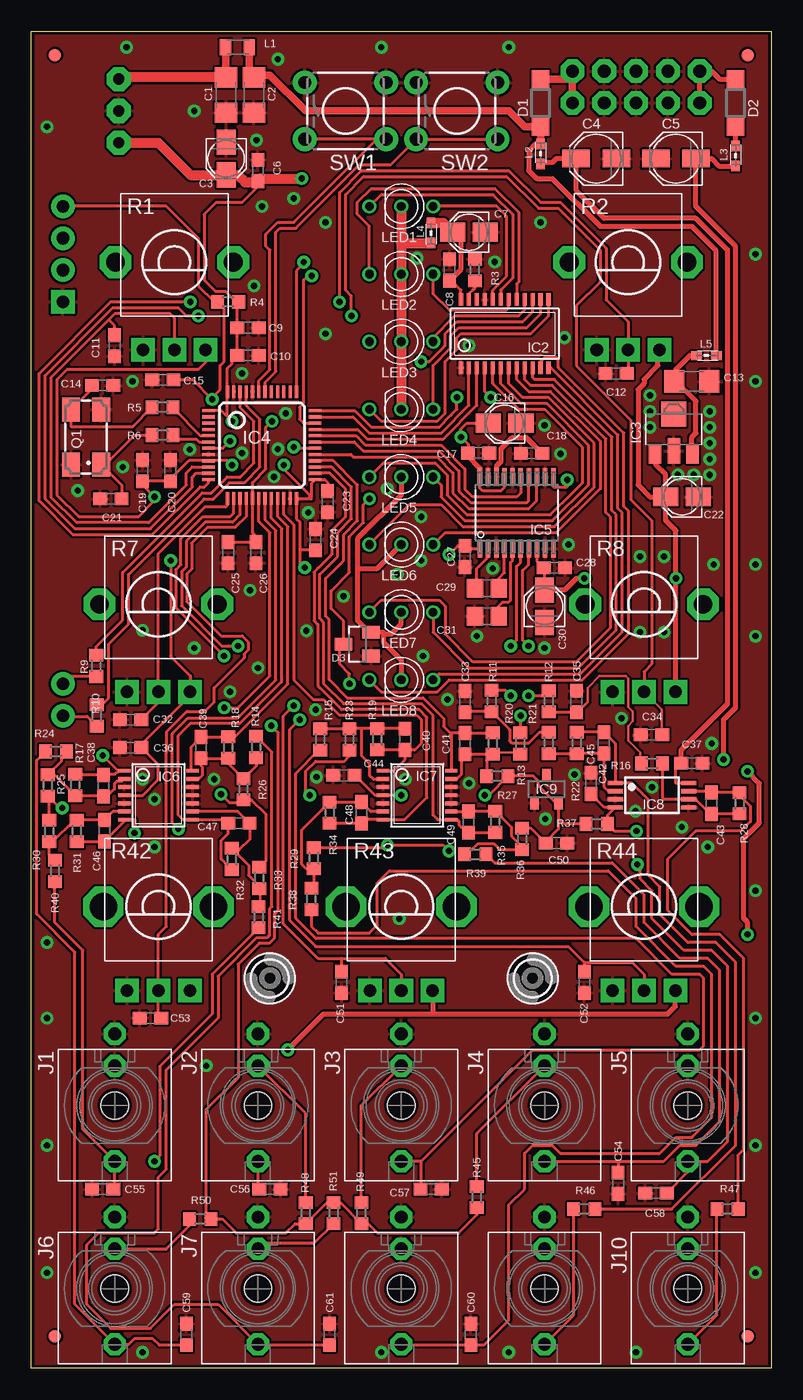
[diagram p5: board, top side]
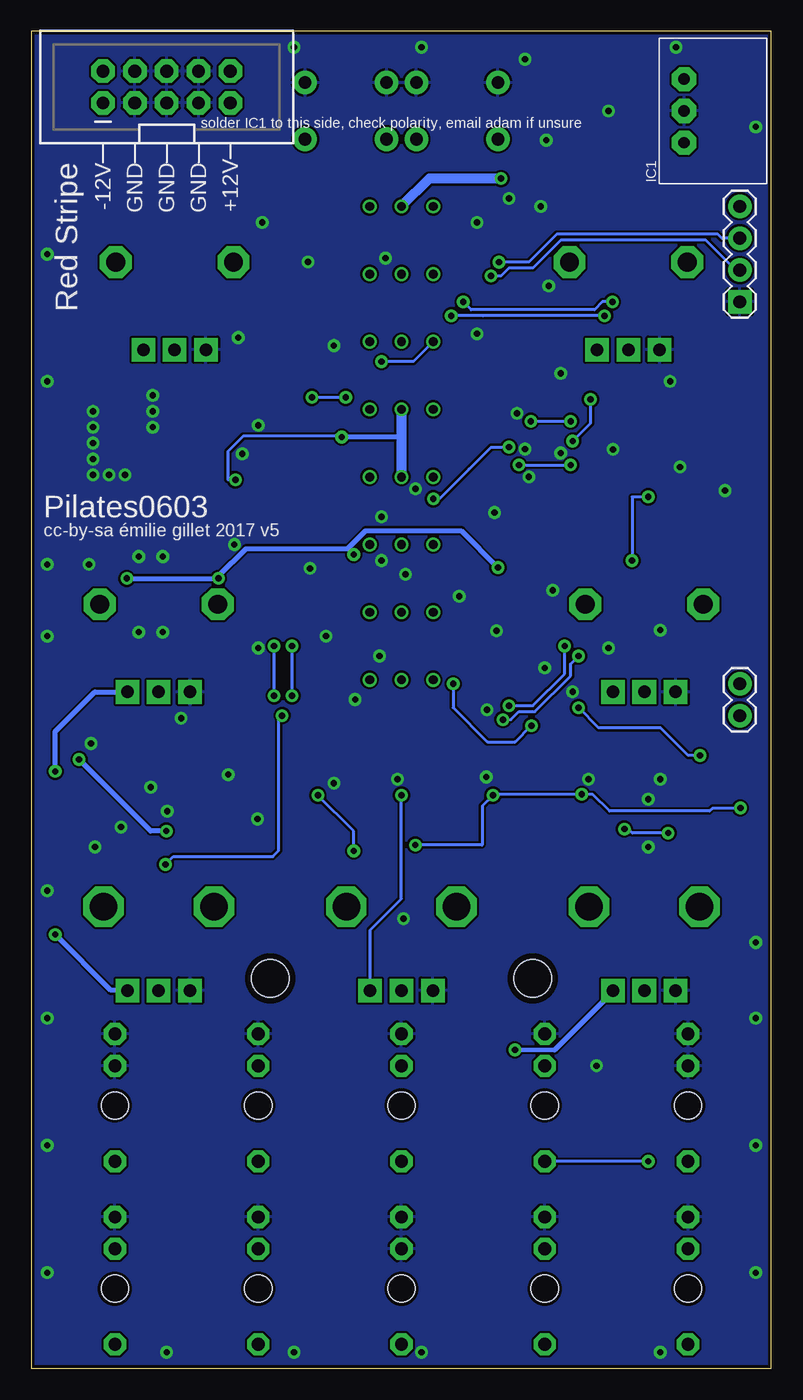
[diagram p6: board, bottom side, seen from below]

Size 59.03 x 106.68 mm. Coordinates in mm from the lower left corner, seen from the top.
Outline: 59.03,0 0,0 0,106.68 59.03,106.68 59.03,0
Copper layers (1*16): Top 0.035mm / dielectric 1.5mm / Bottom 0.035mm
Design rules "PCBCart-Standard *": minimum track width 8mil, minimum drill 0.4mm, track to track 7mil, track to pad 7mil, pad to pad 7mil, via to via 7mil, smd to smd 7mil, copper to edge 10mil, drill to drill 8mil, minimum pad ring 8mil, minimum via ring 10mil, stop-mask expansion 3mil, vias tented up to drill 25mil, thermal gap 8mil

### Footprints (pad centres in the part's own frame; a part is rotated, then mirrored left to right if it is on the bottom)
C1206 = smd 1.6 x 1.8: 1 -1.4,0; 2 1.4,0
PANASONIC_A = smd 2 x 1.5: + 1.3,0; - -1.3,0
PANASONIC_B = smd 2.2 x 1.4: + 1.6,0; - -1.6,0
C0603 = smd 1.1 x 1: 1 -0.85,0; 2 0.85,0
C0805 = smd 1.3 x 1.5: 1 -0.95,0; 2 0.95,0
SOD123 = smd 1.4 x 1.4: A 1.9,0; C -1.9,0
SOT23 = smd 1 x 1.4: 1 -0.95,-1.1; 2 0.95,-1.1; 3 0,1.1
3,0TINY = hole 3: 0,0
WE78 = drill 0.9 pad 1.93 octagon: 1 -2.54,0; 2 0,0; 3 2.54,0
TSSOP24_0635 = smd 0.33 x 1: 1 -3.493,-2.725; 2 -2.857,-2.725; 3 -2.223,-2.725; 4 -1.587,-2.725; 5 -0.953,-2.725; 6 -0.318,-2.725; 7 0.318,-2.725; 8 0.953,-2.725; 9 1.587,-2.725; 10 2.223,-2.725; 11 2.857,-2.725; 12 3.493,-2.725; 13 3.493,2.725; 14 2.857,2.725; 15 2.223,2.725; 16 1.587,2.725; 17 0.953,2.725; 18 0.318,2.725; 19 -0.318,2.725; 20 -0.953,2.725; 21 -1.587,2.725; 22 -2.223,2.725; 23 -2.857,2.725; 24 -3.493,2.725
SOT89 = smd 1 x 1.5: 1 -1.499,-1.981; 3 1.499,-1.981 | smd 1 x 2: 2 0,-1.727 | smd 2 x 2: 2@1 0,1.194
LQFP48 = smd 0.254 x 1: 1 -2.75,-4.25; 2 -2.25,-4.25; 3 -1.75,-4.25; 4 -1.25,-4.25; 5 -0.75,-4.25; 6 -0.25,-4.25; 7 0.25,-4.25; 8 0.75,-4.25; 9 1.25,-4.25; 10 1.75,-4.25; 11 2.25,-4.25; 12 2.75,-4.25; 25 2.75,4.25; 26 2.25,4.25; 27 1.75,4.25; 28 1.25,4.25; 29 0.75,4.25; 30 0.25,4.25; 31 -0.25,4.25; 32 -0.75,4.25; 33 -1.25,4.25; 34 -1.75,4.25; 35 -2.25,4.25; 36 -2.75,4.25 | smd 1 x 0.254: 13 4.25,-2.75; 14 4.25,-2.25; 15 4.25,-1.75; 16 4.25,-1.25; 17 4.25,-0.75; 18 4.25,-0.25; 19 4.25,0.25; 20 4.25,0.75; 21 4.25,1.25; 22 4.25,1.75; 23 4.25,2.25; 24 4.25,2.75; 37 -4.25,2.75; 38 -4.25,2.25; 39 -4.25,1.75; 40 -4.25,1.25; 41 -4.25,0.75; 42 -4.25,0.25; 43 -4.25,-0.25; 44 -4.25,-0.75; 45 -4.25,-1.25; 46 -4.25,-1.75; 47 -4.25,-2.25; 48 -4.25,-2.75
SSOP20 = smd 1.422 x 0.356: 1 -2.845,2.936; 2 -2.845,2.276; 3 -2.845,1.615; 4 -2.845,0.98; 5 -2.845,0.32; 6 -2.845,-0.315; 7 -2.845,-0.98; 8 -2.845,-1.615; 9 -2.845,-2.276; 10 -2.845,-2.936; 11 2.845,-2.936; 12 2.845,-2.276; 13 2.845,-1.615; 14 2.845,-0.98; 15 2.845,-0.315; 16 2.845,0.32; 17 2.845,0.98; 18 2.845,1.615; 19 2.845,2.276; 20 2.845,2.936
TSSOP14_065 = smd 0.305 x 0.991: 1 -1.95,-2.718; 2 -1.3,-2.718; 3 -0.65,-2.718; 4 0,-2.718; 5 0.65,-2.718; 6 1.3,-2.718; 7 1.95,-2.718; 8 1.95,2.718; 9 1.3,2.718; 10 0.65,2.718; 11 0,2.718; 12 -0.65,2.718; 13 -1.3,2.718; 14 -1.95,2.718
TSSOP08 = smd 0.35 x 1.2: 1 -0.975,-2.925; 2 -0.325,-2.925; 3 0.325,-2.925; 4 0.975,-2.925; 5 0.975,2.925; 6 0.325,2.925; 7 -0.325,2.925; 8 -0.975,2.925
DBZ_R-PDSO-G3 = smd 0.7 x 1: 1 -0.95,-1.1; 2 0.95,-1.1; 3 0,1.1
WQP_PJ_301M6 = drill 1.016 pad 1.778 octagon: P1 0,-5.715; P2 0,-3.175; P3 0,4.445 | hole 2.2: 0,0
FIDUCIAL-1X2 = smd 1 x 1: 1 0,0
1X02 = drill 1.016 pad 1.88: 1 0,0; 2 2.54,0
1X04 = drill 1.016 pad 1.88 square: 1 0,0 | drill 1.016 pad 1.88: 2 2.54,0; 3 5.08,0; 4 7.62,0
2X5-SHROUDED = drill 1.016 pad 1.88 octagon: 1 -1.27,5.08; 2 1.27,5.08; 3 -1.27,2.54; 4 1.27,2.54; 5 -1.27,0; 6 1.27,0; 7 -1.27,-2.54; 8 1.27,-2.54; 9 -1.27,-5.08; 10 1.27,-5.08
L2012C = smd 0.9 x 1.25: 1 -0.9,0; 2 1,0
0603 = smd 0.85 x 0.7: 1 -0.9,0; 2 0.7,0
LED-BICOLOR-THROUGHHOLE-LUMEX = drill 0.7: A 0,0; GREEN_C 2.54,0; RED_C -2.54,0
CTS406 = smd 1.9 x 1.4: 1 -2.2,-1.2; 2 2.2,-1.2; 3 2.2,1.2; 4 -2.2,1.2
ALPS_POT_VERTICAL_PS = drill 1 pad 1.88 square: P$1 -2.5,7; P$2 0,7; P$3 2.5,7 | drill 1.5 pad 2.54 octagon: P$4 -4.7,0; P$5 4.7,0
R0603 = smd 1 x 1.1: 1 -0.85,0; 2 0.85,0
ALPS_POT_VERTICAL = drill 1 pad 1.88 square: P$1 -2.5,6.7; P$2 0,6.7; P$3 2.5,6.7 | drill 2.2 pad 3.175 octagon: P$4 -4.4,0; P$5 4.4,0
TACTILE-PTH = drill 1.016 pad 1.88: 1 -3.251,2.261; 2 3.251,2.261; 3 -3.251,-2.261; 4 3.251,-2.261

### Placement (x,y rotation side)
C1  15.54,101.6 270 top
C2  17.76,101.6 270 top
C3  15.54,96.52 270 top
C4  45.06,96.52 180 top
C5  51.41,96.52 180 top
C6  18.08,95.57 90 top
C7  34.91,90.65 180 top
C8  33.36,87.64 90 top
C9  17.28,83.03 0 top
C10  17.28,80.8 0 top
C11  6.65,81.6 270 top
C12  46.65,79.38 180 top
C13  52.68,78.74 0 top
C14  5.7,78.42 180 top
C15  10.49,78.87 180 top
C16  37.76,75.41 180 top
C17  35.69,73.03 0 top
C18  39.91,73 180 top
C19  8.87,71.62 90 top
C20  11.09,71.62 90 top
C21  6.34,69.37 0 top
C22  51.89,69.53 180 top
C23  23.63,69.15 270 top
C24  22.68,66.12 90 top
C25  15.7,65.08 270 top
C26  17.92,65.08 270 top
C27  34.59,64.77 270 top
C28  41.72,63.86 0 top
C29  36.33,62.23 0 top
C30  40.94,60.8 90 top
C31  36.33,60.01 180 top
C32  7.92,51.75 180 top
C33  34.6,53.19 90 top
C34  49.47,50.55 180 top
C35  43.47,53.2 90 top
C36  7.92,49.53 180 top
C37  52.68,48.26 0 top
C38  5.77,46.48 90 top
C39  13.54,49.52 90 top
C40  29.82,50.18 270 top
C41  34.59,49.85 90 top
C42  45.67,49.9 90 top
C43  54.27,45.09 90 top
C44  24.93,47.31 180 top
C45  44.65,46.66 270 top
C46  5.82,42.89 270 top
C47  16.55,43.48 180 top
C48  26.33,44.32 270 top
C49  34.88,43.59 270 top
C50  41.89,41.91 0 top
C51  24.75,30.8 270 top
C52  44.11,30.8 270 top
C53  9.51,27.94 180 top
C54  46.81,14.76 270 top
C55  5.7,14.29 180 top
C56  19.03,14.29 0 top
C57  31.89,14.29 0 top
C58  49.83,13.97 180 top
C59  12.36,2.7 90 top
C60  35.06,2.7 90 top
C61  23.79,2.7 90 top
D1  40.62,100.97 90 top
D2  56.18,100.97 270 top
D3  26,57.78 90 top
H2  39.98,31.12 0 top
H3  19.03,31.11 0 top
IC1  6.97,100.33 270 bottom
IC2  37.76,82.55 0 top
IC3  51.26,74.93 0 top
IC4  18.39,73.66 270 top
IC5  38.72,68.26 90 top
IC6  10.14,45.72 270 top
IC7  30.78,45.72 270 top
IC8  49.51,45.72 270 top
IC9  41.1,46.2 0 top
J1  6.65,20.95 180 top
J2  18.08,20.95 180 top
J3  29.51,20.95 180 top
J4  40.94,20.95 180 top
J5  52.37,20.95 180 top
J6  6.65,6.35 180 top
J7  18.08,6.35 180 top
J8  29.51,6.35 180 top
J9  40.94,6.35 180 top
J10  52.37,6.35 180 top
JP1  1.89,104.78 0 top
JP2  57.13,104.78 0 top
JP3  1.89,2.54 0 top
JP4  57.13,2.54 0 top
JP5  2.52,54.61 270 bottom
JP6  2.52,85.09 90 bottom
JP8  48.24,102.23 90 bottom
L1  16.49,105.41 180 top
L2  40.62,97 90 top
L3  56.18,96.84 90 top
L4  31.89,90.49 270 top
L5  53.95,80.8 0 top
LED1  29.51,92.71 0 top
LED2  29.51,87.31 0 top
LED3  29.51,81.92 0 top
LED4  29.51,76.52 0 top
LED5  29.51,71.12 0 top
LED6  29.51,65.72 0 top
LED7  29.51,60.33 0 top
LED8  29.51,54.93 0 top
Q1  4.38,74.3 90 top
R1  11.41,88.27 180 top
R2  47.6,88.27 180 top
R3  35.39,87.63 90 top
R4  15.7,85.09 180 top
R5  10.46,76.68 180 top
R6  10.46,74.45 180 top
R7  10.14,60.96 180 top
R8  48.88,60.96 180 top
R9  5.17,56.05 90 top
R10  5.22,52.09 90 top
R11  36.71,53.24 90 top
R12  41.28,53.23 90 top
R13  39.01,49.85 90 top
R14  17.93,49.57 90 top
R15  23.04,50.16 270 top
R16  49.51,48.26 180 top
R17  3.51,46.53 270 top
R18  15.7,49.53 270 top
R19  27.6,50.19 90 top
R20  36.81,49.85 270 top
R21  41.27,49.9 90 top
R22  43.52,49.9 270 top
R23  25.38,50.16 270 top
R24  1.96,49.21 180 top
R25  1.31,46.51 270 top
R26  16.92,46.2 270 top
R27  37.17,47.24 0 top
R28  56.49,45.09 270 top
R29  22.54,40.69 90 top
R30  1.43,42.86 90 top
R31  3.62,42.86 90 top
R32  15.99,40.63 90 top
R33  18.19,39.12 90 top
R34  23.79,44.32 90 top
R35  37.01,43.6 90 top
R36  39.15,42.23 90 top
R37  45.11,43.43 180 top
R38  22.34,37.44 270 top
R39  35.41,41.01 0 top
R40  1.89,39.69 270 top
R41  18.13,35.99 270 top
R42  10.14,36.83 180 top
R43  29.51,36.83 180 top
R44  48.88,36.83 180 top
R45  35.54,13.65 270 top
R46  44.11,12.7 0 top
R47  55.54,12.7 0 top
R48  21.89,12.38 270 top
R49  26.33,12.38 270 top
R50  13.47,11.91 180 top
R51  24.11,12.38 90 top
SW1  25.06,100.33 0 top
SW2  33.95,100.33 0 top

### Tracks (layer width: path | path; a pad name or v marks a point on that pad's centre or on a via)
+3V3  (via drill 0.5)
  Top 0.203: 16.17,80.77 16.36,80.77 C10.1 16.17,80.77 | 16.17,80.77 16.05,80.8
  Top 0.254: IC5.17 37.76,71.08 37.76,70.33 37.45,70.01 36.02,70.01 35.78,70.25 IC5.20 | C25.1 C26.1 17.92,66.36 17.64,66.63 IC4.17 17.64,70.69 18.71,71.75 18.71,75.09 v19.19,75.56 | 15.64,75.93 IC4.48 15.64,79.8 16.01,80.17 16.01,80.77 16.05,80.8 | C16.+ 34.75,75.41 34.27,74.93 v34.27,74.3 34.84,73.73 C17.1 | C6.1 18.08,94.3 16.81,93.03 14.74,93.03 13.79,92.08 13.79,86.84 14.68,85.94 15.47,85.94 15.65,85.77 15.65,85.76 16.43,84.98 | 15.64,75.93 15.17,76.41 IC4.1 | C10.1 C9.1 | C9.1 | C9.1 16.43,84.98 | R4.1 16.43,84.98 | IC5.11 41.65,70.37 41.74,70.28 42.65,70.28 42.75,70.38 v42.75,70.89 | v16.01,75.56 | v16.01,75.56 15.64,75.93
  Top 0.406: LED5.A 29.51,69.69 26.02,66.2 26.02,63.82 | LED6.A 27.6,63.82 26.02,63.82 | 26.02,63.82 26.02,59.69 26.98,58.73 D3.2 28.08,58.73 28.08,58.58 | LED7.A 29.51,59.37 28.71,58.58 28.08,58.58 | LED8.A 29.51,56.52 28.08,57.94 28.08,58.58 | IC5.20 35.78,71.83 34.84,72.78 C17.1
  Top 0.813: LED4.A LED3.A LED2.A 29.51,89.79 | 29.51,89.79 L4.2 | LED1.A 29.51,89.79 | v21.57,94.93 18.29,94.93 C6.1 18,94.64 17.05,94.64 16.47,95.22 C3.+ 12.71,95.22 10.14,97.79 IC1.3
  Bottom 0.254: v19.19,75.56 v16.01,75.56 | v34.27,74.3 34.35,74.37 42.14,74.37 43.36,73.15 43.36,70.89 v42.75,70.89
  Bottom 0.406: 29.51,74.3 v34.27,74.3
  Bottom 0.813: LED4.A 29.51,74.3 LED5.A | LED1.A 27.29,94.93 v21.57,94.93
+3V3_A  (via drill 0.5)
  Top 0.203: 34.65,65.42 34.65,65.53 C27.1
  Top 0.254: 22.36,69.53 20.14,71.75 v20.14,72.07 | v16.01,72.07 15.68,72.41 IC4.9 12.54,72.41 11.09,70.96 C20.1 C19.1 8.87,70.48 v9.82,69.53 9.82,69.22 8.55,67.94 3.79,67.94 2.04,69.69 2.04,78.9 2.84,79.69 13.32,79.69 13.91,80.29 R1.P$1 | R7.P$1 12.64,53.66 | 22.36,69.53 22.36,70.63 IC4.25 23.41,70.91 23.63,70.68 C23.1 | 34.65,65.42 IC5.1 | v33.32,64.93 34.01,65.62 C27.1 | IC6.4 8.87,45.72 10.14,46.99 10.14,48.16 C36.1 8.77,49.78 12.64,53.66 | C44.1 25.84,47.31 27.43,45.72 IC7.4 v29.51,45.72 | 22.36,69.53 22.21,69.53 22.36,69.37 21.34,69.37 21.26,69.29 IC4.24 21.14,67.77 21.44,67.48 21.44,65.27 | 21.44,65.27 21.44,64.06 21.62,63.89 v21.81,63.89 | C30.+ 40.94,63.8 C28.1 40.33,64.41 IC5.8 | C24.1 21.44,65.27 | v11.12,64.45 11.12,56.81 12.68,55.24 12.68,53.7 12.64,53.66
  Top 0.406: R8.P$1 51.41,54 v51.41,63.02 51.41,66.83 50.59,67.66 C22.+ | 32.05,28.26 23.32,28.26 v20.46,25.4 | 32.05,28.26 50.78,28.26 51.38,28.85 R44.P$1 | R43.P$1 32.05,30.09 32.05,28.26 | v57.13,34.61 57.13,35.56 56.81,35.88 56.81,42.25 58.08,43.52 58.08,46.67 v57.13,47.62 | C30.+ 42.55,62.1 43.48,63.02 v44.11,63.02 | R2.P$1 49.99,81.15 49.99,80.01 48.88,78.9 48.88,78.58 48.4,78.11 48.4,70.48 49.35,69.53 C22.+ | IC3.1 49.83,72.95 49.83,72.07 50.59,71.31 C22.+
  Bottom 0.254: 33.79,65.41 v33.32,64.93 | v11.12,64.45 11.12,69.53 v9.82,69.53 | v29.51,45.72 29.51,37.47 32.01,34.97 R43.P$1 | v20.14,72.07 v16.01,72.07
  Bottom 0.356: 17.28,25.4 v20.46,25.4
  Bottom 0.406: v51.41,63.02 v44.11,63.02 44.11,63.19 41.9,65.41 33.79,65.41 32.36,66.83 24.75,66.83 v21.81,63.9 v21.81,63.89 | R44.P$1 51.41,30.16 52.68,30.16 v57.13,34.61 | v57.13,47.62 57.13,50.8 53.97,53.96 R8.P$1 | 17.28,25.4 12.64,30.04 R42.P$1
ADC_FM
  Top 0.254: IC4.22 20.14,68.1 20.93,67.31 20.93,54.93 22.51,53.35 23.33,53.35 24.57,52.11 30.73,52.11 31.09,51.75 31.09,49.85 30.57,49.33 C40.2 | IC7.1 28.92,47.67 29.82,48.58 C40.2 | C40.2 27.62,49.33 R19.1
ADC_GATE
  Top 0.254: IC4.21 19.64,67.97 20.46,67.15 20.46,54.61 16.23,50.38 R18.1 15.69,50.37 C39.2 12.74,49.56 12.74,47.79 IC6.14
ADC_HARMONICS
  Top 0.254: R20.1 C41.2 33.63,50.7 | IC4.28 24.09,72.41 26.02,70.48 26.02,67.63 24.9,66.52 24.9,64.45 23.48,63.02 23.48,60.02 23.75,59.74 23.75,54.95 25.21,53.5 31.25,53.5 32.89,51.86 32.89,51.23 33.42,50.7 33.63,50.7 | 33.63,50.7 33.49,50.56 IC7.14
ADC_MODEL  (via drill 0.5)
  Top 0.254: v11.73,43.02 11.25,43.5 11.25,50.64 12.49,51.88 16.46,51.88 19.51,54.93 19.51,66.83 18.64,67.69 IC4.19 | v8.24,42.7 8.24,43.77 IC6.7 7.42,43.64 C46.2 5.8,42.01 R31.1
  Bottom 0.254: v8.24,42.7 11.09,42.7 11.41,43.02 v11.73,43.02
ADC_MORPH
  Top 0.254: R35.1 34.89,42.75 C49.2 34.86,42.74 34.42,43.17 34.28,43.17 34.1,43.35 34.1,43.67 34,43.77 IC7.8 32.41,43.77 32.05,44.13 32.05,52.07 31.09,53.02 24.9,53.02 23.29,54.64 23.29,59.54 23.16,59.67 23.16,59.69 23,59.85 23,63.34 24.43,64.77 24.43,66.67 25.54,67.79 25.54,70.33 23.96,71.91 IC4.27
ADC_TIMBRE
  Top 0.254: IC4.20 19.14,67.83 19.98,66.99 19.98,54.93 19.94,54.88 19.94,54.75 16.62,51.44 12.68,51.44 11.73,50.48 11.73,44.13 12.09,43.77 IC6.8 15.42,43.77 C47.2 15.7,42.67 15.14,42.1 15.14,40.63 R32.1
ADC_TRIG  (via drill 0.5)
  Top 0.254: 6.92,47.67 v5.7,48.9 | IC4.18 18.14,67.56 19.03,66.67 19.03,55.24 16.47,52.68 16.02,52.68 16,52.7 v15.38,52.7 | R17.1 5.72,47.38 | IC6.1 6.92,47.67 | C38.2 5.72,47.38 | 6.92,47.67 6.63,47.38 5.72,47.38
  Bottom 0.254: v5.7,48.9 6.65,48.9 8.85,51.09 13.77,51.09 v15.38,52.7
ADC_V_OCT
  Top 0.254: IC4.26 23.82,71.41 25.06,70.17 25.06,67.94 23.95,66.83 23.95,64.93 22.84,63.82 22.84,63.79 22.57,63.52 22.57,59.65 22.86,59.36 22.86,54.45 22.99,54.31 22.99,54.3 24.75,52.55 30.94,52.55 31.55,51.93 31.55,45.54 29.78,43.77 IC7.7 26.63,43.77 C48.2 R34.1
AREF_-10  (via drill 0.5)
  Top 0.254: R30.2 1.43,45.54 R25.2 2.27,44.7 v2.47,44.7 | 15.79,45.14 16.71,45.14 R26.2 17.56,45.35 18.69,44.22 18.69,40.46 R33.2 | R23.2 25.38,48.84 24.97,48.43 22.67,48.43 21.89,47.65 21.89,46.04 v22.21,45.72 | v36.17,45.72 36.49,45.72 R27.2 40.06,47.24 40.44,46.86 40.44,46.51 41.85,45.1 IC9.2 42.05,43.87 | v33.32,41.27 32.85,41.74 v28.4,41.74 28.2,41.54 R29.2 | v15.13,45.8 15.79,45.14 | 15.79,45.14 | R36.2 39.2,43.08 39.22,43.05 39.9,43.05 40.99,41.96 | C50.1 40.99,41.96 | 42.05,43.87 42.05,43.02 40.99,41.96 | R37.2 42.48,43.43 42.05,43.87
  Bottom 0.254: v33.32,41.27 33.32,42.86 v36.17,45.72 | v2.47,44.7 4.69,44.7 4.95,44.45 12.91,44.45 14.26,45.8 v15.13,45.8 22.13,45.8 v22.21,45.72 23.05,44.87 23.05,41.78 23.09,41.74 v28.4,41.74
DAC_BCK
  Top 0.254: IC5.13 40.3,71.08 40.3,69.22 39.67,68.58 34.9,68.58 33.63,69.85 33.63,71.44 32.36,72.71 25.7,72.71 25.5,72.91 IC4.29
DAC_DIN
  Top 0.254: IC5.14 39.67,71.08 39.67,69.22 39.51,69.06 35.06,69.06 34.11,70.01 34.11,71.6 32.52,73.18 26.49,73.18 25.77,73.91 IC4.31
DAC_LRCK
  Top 0.254: IC5.15 39.03,69.85 38.71,69.53 35.22,69.53 34.59,70.17 34.59,71.75 32.68,73.66 26.65,73.66 | IC4.32 25.9,74.41 26.65,73.66 | 26.65,73.66
FM_IN
  Top 0.254: 31.09,16.51 J3.P3 | 31.09,16.51 39.98,25.4 53.32,25.4 53.64,25.72 53.64,31.11 53.32,31.43 51.1,31.43 48.24,34.29 22.7,34.29 21.1,35.89 21.1,47.47 22.94,49.31 R15.2 | C57.1 31.09,14.34 31.09,16.51
FREQ_ATT  (via drill 0.5)
  Top 0.254: R43.P$2 29.51,31.43 28.24,32.7 24.75,32.7 | C51.1 24.75,32.7 | v20.93,52.86 20.1,52.03 20.1,35.45 22.84,32.7 24.75,32.7 | v16.49,57.63 15.73,57.63 15.71,57.64 15.18,57.64 11.98,60.84 11.98,63.55 12.36,63.93 12.36,66.02 13.86,67.51 16.06,67.51 16.64,68.1 IC4.15
  Bottom 0.254: v20.93,52.86 19.03,52.86 16.49,55.4 v16.49,57.63
FREQ_POT
  Top 0.254: R1.P$2 11.41,83.82 11.09,84.14 6.65,84.14 6.17,83.66 | IC4.10 12.84,71.91 12.36,71.44 12.36,70.48 9.35,67.47 3.63,67.47 1.57,69.53 1.57,79.06 6.17,83.66 | C11.1 6.65,83.19 6.17,83.66
GATE_IN
  Top 0.254: C61.1 18.13,1.85 J7.P3 14.9,5.08 11.41,5.08 9.51,3.17 6.33,3.17 4.43,5.08 4.43,9.84 5.38,10.79 9.82,10.79 10.14,11.11 10.14,15.24 10.78,15.88 10.78,23.81 14.9,27.94 14.9,31.28 17.96,34.34 18.8,34.34 18.98,34.52 18.98,36.63 19.18,36.83 19.18,49.16 R14.2
GATE_IN1
  Top 0.254: C59.1 10.2,1.85 9.66,2.38 8.24,2.38 7.76,1.91 J6.P3 3.47,5.08 3.47,33.18 0.41,36.24 0.41,48.51 R24.2
GND  (via drill 0.5)
  other vias: 30.78,88.58 36.96,88.29 34.9,81.6 36.81,63.82 14.59,47 42.84,65.72 40.94,57.47 35.54,58.42 22.75,47.18 34.9,46.67 43.33,47.37 54.27,49.85 7.29,71.91 27.92,105.41 17.96,97.99 53.95,41.59 49.35,75.09 54.43,64.14 12.64,73.31 3.71,70.03 29.82,46.99 17.44,62.07 19.35,71.12 29.19,63.34 28.4,70.17 21.94,58.85 29.35,35.88 18.08,55.88 15.86,53.98 16.81,79.38 20.3,76.2 9.82,41.59 41,43.83 40.62,91.44 23.48,91.44 13,57.47 8.87,58.9 19.66,73.34 31.09,67.94 31.09,64.45 1.25,7.62 1.25,17.78 1.25,27.94 1.25,33.97 1.25,99.06 7.6,105.41 19.66,104.46 38.08,105.41 57.76,88.9 42.52,82.23 48.56,58.74 57.76,78.74 57.76,64.14 57.76,58.42 57.76,38.1 57.76,27.94 57.76,17.78 57.76,7.62 8.87,1.27 27.92,1.27 38.08,1.27 48.24,1.27 20.93,93.34 48.56,64.77 50.46,58.74 33.2,53.36 47.08,51.87 17.76,86.36 18.39,92.71 16.81,73.03 51.89,43.18 49.51,46.35 8.08,78.74 13,100.33 22.68,52.55 8.87,46.99 9.82,45.4 13.95,24.13 40.94,75.25 42.21,72.96 50.46,64.77 23.48,82.55 31.25,56.83 24.9,61.59 49.35,76.36 54.11,75.09 54.11,73.82 54.11,76.36 49.35,77.63 54.11,72.55 54.11,71.28 52.84,71.28 51.57,71.28 22.08,68.28 48.2,44.45
  pour Top: 59.03,106.68 59.03,0 -0.02,0 -0.02,106.68
  pour Bottom: 59.03,106.68 59.03,0 -0.02,0 -0.02,106.68
HARMONICS_IN  (via drill 0.5)
  Top 0.254: C58.1 52.37,15.66 J5.P3 53.95,16.51 55.54,18.1 55.54,32.07 54.27,33.34 52.05,33.34 49.51,35.88 49.51,38.1 48.56,39.05 48.56,39.98 v48.34,40.2 | R13.2 39.03,50.72 v39.03,52.07
  Bottom 0.254: v39.03,52.07 39.3,51.8 39.3,41.3 39.77,40.83 47.71,40.83 v48.34,40.2
HARMONICS_POT  (via drill 0.5)
  Top 0.254: IC4.12 14.14,70.68 13.79,70.33 13.47,70.33 9.66,66.52 3.31,66.52 0.61,69.22 0.61,79.38 6.33,85.09 v12.68,85.09 | v24.59,85.09 24.59,93.82 26.33,95.57 38.08,95.57 40.62,93.03 42.21,93.03 45.86,89.38 45.86,85.25 47.6,83.5 R2.P$2 47.6,79.48 C12.1
  Bottom 0.254: v12.68,85.09 13.47,85.09 14.11,84.45 23.95,84.45 v24.59,85.09
LEDS_SCK
  Top 0.254: IC4.33 26.04,74.91 26.81,74.14 32.84,74.14 35.54,76.83 IC2.3
LEDS_SIN
  Top 0.254: IC4.35 25.67,75.91 26.97,74.61 32.68,74.61 34.9,76.83 IC2.2
LEDS_SS  (via drill 0.5)
  Top 0.254: 26.65,75.56 27.13,75.09 32.52,75.09 33.48,76.04 | 26.65,75.56 | 26.65,75.56 25.8,76.41 IC4.36 | 33.48,76.04 | 33.48,76.04 33.95,76.52 v33.95,77.47 | v36.65,77.47 36.17,77.95 IC2.4
  Bottom 0.254: v33.95,77.47 v36.65,77.47
MODEL_IN
  Top 0.254: R40.2 1.89,35.56 4.11,33.34 4.11,19.05 J1.P3 6.65,14.39 C55.1
MORPH_ATT  (via drill 0.5)
  Top 0.254: R44.P$2 48.88,31.43 47.92,32.38 44.11,32.38 | 44.11,32.38 C52.1 | IC4.14 16.14,68.23 15.86,67.94 13.68,67.94 11.93,66.19 11.93,64.11 11.55,63.73 11.55,60.66 v15.38,56.83 | v21.41,51.75 20.62,50.97 20.62,35.71 22.68,33.66 42.84,33.66 44.11,32.38
  Bottom 0.254: v15.38,56.83 | v15.38,56.83 16.01,56.2 16.01,55.24 18.87,52.39 20.14,52.39 20.78,51.75 v21.41,51.75
MORPH_IN
  Top 0.254: J4.P3 46.81,16.51 | 46.81,16.51 50.46,16.51 51.73,17.78 53,17.78 54.91,19.68 54.91,31.75 53.95,32.7 51.73,32.7 48.88,35.56 48.88,37.78 46.33,40.32 36.95,40.32 R39.2 | C54.1 | 46.81,16.51 C54.1
MORPH_POT  (via drill 0.5)
  Top 0.203: C34.1 50.27,50.67 50.27,52.58 48.94,53.91 R8.P$2
  Top 0.254: R8.P$2 48.88,55.56 49.51,56.2 49.51,67.63 47.83,69.3 47.83,75.65 43.48,80.01 43.48,84.77 45.38,86.68 45.38,89.22 42.05,92.55 40.46,92.55 37.92,95.09 26.49,95.09 25.06,93.66 25.06,86.04 25.54,85.57 v25.54,83.98 | IC4.11 13.13,71.41 12.84,71.12 12.84,70.33 9.51,66.99 3.47,66.99 1.09,69.37 1.09,79.22 6.49,84.61 11.73,84.61 12.36,83.98 v13.32,83.98
  Bottom 0.254: v13.32,83.98 23,83.98 | 23,83.98 | 23,83.98 v25.54,83.98
N$1
  Top 0.61: 15.49,103.05 L1.2
  Top 0.813: 15.49,103.05 C1.1 7.1,103 IC1.1
N$2
  Top 0.254: 45.06,56.67 47.13,58.74 47.13,68.26 46.79,68.6 46.79,74.47 41.44,79.83 IC2.12 | 45.06,56.67 | 45.06,56.67 43.79,55.4 32.52,55.4 LED8.GREEN_C
N$3
  Top 0.203: 12.81,11.56 12.74,11.62 12.74,11.81 R50.2
  Top 0.254: J6.P2 10.78,9.53 12.81,11.56
N$4
  Top 0.254: IC6.2 7.23,46.83 6.8,46.83 6.62,46.65 6.62,46.22 6.03,45.63 C38.1 5.72,45.68 R17.2 1.84,47.36 R25.1 2.37,48.41 2.37,48.77 R24.1
N$5
  Top 0.254: LED8.RED_C 27.92,53.98 32.36,53.98 33.32,54.93 43.95,54.93 47.6,58.58 47.6,68.42 47.27,68.76 47.27,74.63 42.05,79.85 42.05,80.49 41.89,80.64 40.94,80.64 40.62,80.33 IC2.11
N$6
  Top 0.254: C29.1 35.54,62.39 35.54,63.82 36.44,64.72 IC5.2
N$7
  Top 0.254: IC4.5 13.49,74.41 11.31,76.6 R5.1
N$8
  Top 0.254: IC4.6 13.38,73.91 13.16,74.14 11.62,74.14 R6.1
N$9
  Top 0.254: IC2.10 39.98,79.06 40.14,78.9 41.73,78.9 46.32,74.31 46.32,68.44 46.65,68.1 46.65,58.9 43.64,55.88 34.9,55.88 32.05,58.74 LED7.GREEN_C
N$10
  Top 0.254: LED7.RED_C 27.92,61.28 32.52,61.28 33,60.8 33,58.58 35.22,56.36 43.48,56.36 46.18,59.05 46.18,67.94 45.84,68.28 45.84,74.16 41.57,78.42 39.83,78.42 39.35,78.9 IC2.9
N$11
  Top 0.254: LED6.GREEN_C 33,66.67 41.89,66.67 45.39,70.17 45.39,73.97 41.41,77.95 39.67,77.95 38.71,78.9 IC2.8
N$12
  Top 0.254: IC2.13 41.25,83.98 39.83,82.55 34.27,82.55 33.95,82.23 33.95,81.28 33,80.33 33,76.2 32.36,75.56 27.92,75.56 LED4.RED_C
N$13
  Top 0.254: LED6.RED_C 30.14,68.9 32.68,68.9 34.43,67.15 41.73,67.15 44.89,70.31 44.89,73.84 41.25,77.47 39.19,77.47 38.08,78.58 IC2.7
N$14
  Top 0.254: LED4.GREEN_C 32.05,80.01 33.48,81.44 33.48,82.39 34.11,83.03 39.51,83.03 40.62,84.14 IC2.14
N$15
  Top 0.254: LED5.GREEN_C 32.68,70.48 32.68,69.53 34.59,67.63 41.57,67.63 44.41,70.47 44.41,73.68 41.1,76.99 39.03,76.99 37.45,78.58 IC2.6
N$16
  Top 0.254: C29.2 37.29,63.02 37.73,63.47 IC5.4
N$17  (via drill 0.5)
  Top 0.254: v31.09,80.33 31.73,80.33 33,81.6 33,82.55 33.95,83.5 39.19,83.5 39.98,84.3 IC2.15
  Bottom 0.254: v31.09,80.33 28.55,80.33 LED3.RED_C
N$18
  Top 0.254: LED3.GREEN_C 32.05,82.23 33.79,83.98 38.87,83.98 39.35,84.45 IC2.16
N$19
  Top 0.254: LED2.RED_C 26.97,91.12 26.02,92.08 26.02,93.03 27.13,94.14 36.97,94.14 38.87,92.23 38.87,86.68 38.71,86.52 IC2.17
N$20
  Top 0.254: LED2.GREEN_C 32.05,85.72 33.32,84.45 37.92,84.45 38.08,84.61 IC2.18
N$21
  Top 0.254: LED1.RED_C 27.92,93.66 36.81,93.66 38.4,92.08 38.4,87 37.45,86.04 IC2.19
N$22
  Top 0.254: 43.16,69.85 41.41,68.1 34.75,68.1 33.16,69.69 33.16,71.28 32.21,72.23 28.08,72.23 LED5.RED_C | 43.16,69.85 | 43.16,69.85 43.93,70.62 43.93,73.52 | IC2.5 36.81,78.58 38.87,76.52 40.94,76.52 43.93,73.52 | 43.93,73.52
N$23
  Top 0.254: LED1.GREEN_C 37.13,92.71 37.92,91.92 37.92,87.15 36.81,86.04 IC2.20
N$24
  Top 0.254: J3.P2 26.33,20.95 R49.1
N$25
  Top 0.254: J2.P2 21.89,20.32 R48.1
N$26
  Top 0.254: J4.P2 35.54,18.73 R45.1
N$27
  Top 0.254: IC2.24 34.27,86.04 33.53,86.79 C8.1
  Top 0.406: C8.1 34.28,87.71 34.28,89.97 C7.+
  Top 0.813: C7.+ 32.86,91.39 L4.1
N$28
  Top 0.254: R14.1 17.93,48.06 R26.1 15.7,48.27 R18.2 15.69,48.67 C39.1 13.54,48.06 13.66,47.95 13.66,47.33 13.35,47.02 IC6.13
N$29
  Top 0.254: R5.2 8.07,75.14 3.17,75.14 Q1.3 4.85,78.17 C14.2
N$30
  Top 0.254: IC7.6 27.09,44.42 C48.1 R34.2 21.58,42.96 21.58,40.2 21.94,39.84 R29.1 22.54,38.48 R38.1
N$31  (via drill 0.5)
  Top 0.254: v9.82,16.51 10.3,16.99 10.3,24.13 14.43,28.26 14.43,31.43 R41.2 | C56.1 18.08,14.39 J2.P3
  Bottom 0.254: v9.82,16.51 J2.P3
N$32
  Top 0.254: IC7.9 34.86,44.42 C49.1 34.89,44.45 R35.2 38.29,43.17 38.29,42.45 39.15,41.6 R36.1 37.38,41.38 36.89,41.86 35.64,41.86 35.15,41.38 34.93,41.38 R39.1
N$33
  Top 0.254: JP5.2 2.58,52.01 4.44,52.01 R10.1
N$34
  Top 0.254: C40.1 27.62,51.03 R19.2 26.33,51.04 | 26.33,51.04 25.41,51.04 R23.1 R15.1 | 26.33,51.04 26.33,48.9 26.97,48.26 26.97,47.31 27.25,47.02 IC7.2
N$35
  Top 0.254: R6.2 8.24,74.45 5.88,72.1 Q1.1 7.19,70.48 C21.2
N$36
  Top 0.254: J7.P2 18.5,9.95 22.52,9.95 R51.1
N$37
  Top 0.254: IC6.6 6.5,44.42 C46.1 3.65,43.74 R31.2 3.42,43.71 1.72,42.01 R30.1 1.43,40.99 R40.1
N$38
  Top 0.406: L3.2 D2.A
N$39
  Top 0.203: 16.55,41.34 16.36,41.15 R32.2 | R33.1 18.27,38.1 18.27,36.96 R41.1
  Top 0.254: IC6.9 16.47,44.42 C47.1 17.4,42.19 16.55,41.34 | R32.2 17.34,40.13 17.34,39.34 18.19,38.48 R33.1
N$40
  Top 0.406: L5.2 54.59,80.87 54.59,89.22 52.68,91.12 45.38,91.12 41.57,94.93 40.3,94.93 39.67,95.57 39.67,97.16 40.21,97.7 L2.2
  Top 0.61: L2.2 D1.C 39.34,99.06 38.08,100.33 21.89,100.33 19.03,103.19 17.95,103.19 C2.1 | 17.49,103.27 17.39,103.37 L1.1
  Top 0.813: 17.49,103.27 C2.1
N$41
  Top 0.203: R13.1 38.84,49.15 36.94,49.15 R20.2
  Top 0.254: IC7.13 33.92,47.02 34.29,47.39 34.29,48.7 C41.1 R20.2 36.32,48.5 R27.1
N$42
  Top 0.406: 51.41,78.74 51.41,79.69 52.53,80.8 L5.1 | IC3.3 52.68,73.02 52.68,74.3 53,74.61 53,77.15 51.41,78.74 | 51.41,78.74 C13.1
N$43  (via drill 0.5)
  Top 0.254: IC5.6 39.03,64.29 38.71,63.98 38.71,58.1 v38.24,57.63 | R11.2 37.81,54.09 v38.24,53.66
  Bottom 0.254: v38.24,53.66 v38.24,57.63
N$46
  Top 0.254: C33.1 34.65,52.39 R11.1 38.15,50.95 38.15,50.07 38.33,49.89 39.68,49.89 40.54,50.75 R21.2
N$47
  Top 0.203: 44.37,53.15 44.37,54.29 45.32,55.24 47.41,55.24 47.6,55.05 47.6,52.77 47.99,52.39 47.99,51.63 47.6,51.24 47.6,50.1 48.56,49.15 48.56,48.39 R16.2 | 43.41,52.38 43.41,52.39 C35.1
  Top 0.254: 44.37,53.15 43.57,52.35 C35.1 | R12.1 43.41,52.38
N$48
  Top 0.254: IC5.5 38.4,64.45 38.24,64.29 38.24,61.28 38.08,61.12 37.6,61.12 37.28,60.8 C31.1
N$51
  Top 0.254: JP5.1 2.52,54.66 3.09,55.23 3.12,55.2 R9.1
N$54
  Top 0.406: IC5.18 37.13,71.14 37.13,72.03 37.47,72.37 37.47,73.36 38.38,74.28 39.48,74.28 C18.1
N$55  (via drill 0.5)
  Top 0.254: IC5.7 39.67,65.39 39.67,64.14 39.19,63.66 39.19,58.1 v39.67,57.63 | v39.67,53.66 40.86,53.66 R12.2
  Bottom 0.254: v39.67,53.66 v39.67,57.63
N$56
  Top 0.61: JP8.9 43.16,102.87 | 43.16,102.87 JP8.10 | D1.A 43.16,102.87
N$58
  Top 0.254: R16.1 50.36,45.52 50.48,45.4 IC8.6 53.01,45.4 54.17,44.23 C43.1 R28.2
N$60
  Top 0.203: R28.1 56.56,45.91 56.56,45.72 56.52,45.69
  Top 0.254: R47.2 56.39,17.04 56.81,17.46 56.81,32.7 54.91,34.61 52.68,34.61 50.78,36.51 50.78,40.64 53,42.86 56.6,42.86 57.35,43.61 57.35,44.86 56.52,45.69 | IC8.7 54.16,46.05 C43.2 R28.1
N$62
  Top 0.203: 46.17,46.05 IC8.2
  Top 0.254: R21.1 R22.2 C42.1 45.68,46.39 46.03,46.05 46.17,46.05
N$63
  Top 0.254: R46.2 51.1,12.7 56.18,17.78 56.18,32.38 54.59,33.97 52.37,33.97 50.14,36.2 50.14,38.42 49.19,39.37 49.19,45.4 47.9,46.7 IC8.1 46.58,49.84 C42.2 R22.1
N$64
  Top 0.406: D2.C 54.91,102.87 54.27,103.5 JP8.2 JP8.1
N$65
  Top 0.254: J9.P3 43.26,4.23 R46.1
N$68
  Top 0.254: IC2.23 34.9,85.74 35.25,86.08 35.31,86.08 35.39,86.16 R3.1
N$69
  Top 0.254: J10.P3 54.69,4.23 R47.1
NORMALIZATION_PROBE  (via drill 0.5)
  Top 0.203: 26.08,11.75 26.08,11.81 R49.2 | 13.89,12 14.27,12 R50.1 13.89,12 | 13.89,12 13.95,12.03
  Top 0.254: v26.97,69.37 26.49,68.9 26.49,67.47 25.38,66.36 25.38,63.5 23.91,62.03 23.91,60.61 24.9,59.62 D3.3 24.59,57.46 24.59,56.2 25.38,55.4 v25.38,54.61 | v20.93,73.5 21.03,73.41 IC4.30 | 13.95,12.03 13.95,20.64 16.49,23.18 16.49,32.23 18.17,33.91 18.98,33.91 19.41,34.34 19.41,36.26 19.66,36.51 19.66,50.74 v19.14,51.27 | R50.1 15.22,11.91 16.33,10.79 20.3,10.79 21.04,11.53 R48.2 23.59,13.23 R51.2 24.63,13.23 R49.2 | 26.08,11.75 26.65,11.75 27.6,10.79 34.11,10.79 35.54,12.22 R45.2
  Bottom 0.254: v25.38,54.61 25.38,52.7 22.65,49.98 22.65,49.97 20.43,49.97 v19.14,51.27 | 24.11,71.75 22.36,73.5 v20.93,73.5 | v26.97,69.37 26.49,69.37 24.11,71.75 | 24.11,71.75
RESET  (via drill 0.5)
  Top 0.254: v15.86,73.98 15.29,73.41 IC4.7 | v14.43,77.31 14.43,77.47 15.06,78.11 15.06,80.01 15.38,80.33 15.38,84.56 R4.2 14.59,85.09 13.32,86.36 13.32,90.17 10.78,92.71 JP6.4 | v14.43,77.31 | C15.1 12.86,78.87 v14.43,77.31
  Bottom 0.254: v15.86,73.98 14.43,75.41 v14.43,77.31
RX
  Top 0.254: R9.2 5.17,57.58 7.28,59.69 7.28,63.5 13.63,69.85 14.35,69.85 15.62,71.12 16.65,71.12 17.76,72.23 17.76,75.56 16.64,76.68 IC4.46
SW_1
  Top 0.254: SW1.3 SW1.4 27.56,98.07 20.93,91.44 19.66,91.44 18.71,90.49 18.71,89.53 19.03,89.22 19.03,79.69 18.14,78.81 IC4.43
SW_2
  Top 0.254: SW2.4 SW2.3 28.68,96.04 26.17,96.04 21.09,90.96 19.82,90.96 19.51,90.65 19.51,79.53 19.19,79.22 | IC4.42 18.64,78.67 19.19,79.22 | 19.19,79.22
SWCLK  (via drill 0.5)
  Top 0.203: 21.78,88.21 21.89,88.2 v21.73,88.27
  Top 0.254: 21.78,88.21 21.14,87.58 IC4.37
  Bottom 0.254: v21.73,88.27 19.35,88.27 17.12,90.49 4.27,90.49 3.95,90.17 JP6.3
SWDIO  (via drill 0.5)
  Top 0.254: IC4.34 21.73,75.41 21.41,75.72 21.41,76.68 21.73,76.99 21.73,86.84 22.05,87.15 v22.36,87.15
  Bottom 0.254: v22.36,87.15 21.57,87.15 20.93,87.79 19.03,87.79 16.81,90.01 5.22,90.01 2.84,87.63 JP6.2
TIMBRE_ATT
  Top 0.203: 10.14,28 10.27,28 C53.1
  Top 0.254: 10.14,28 R42.P$2 10.14,34.61 10.78,35.24 10.78,49.16 10.82,49.2 10.82,50.82 12.41,52.41 13.85,52.41 14.59,53.15 14.59,54.29 16.98,56.69 16.98,56.98 17.3,57.29 17.3,57.96 16.82,58.44 15.14,58.44 12.41,61.16 12.41,63.38 12.79,63.75 12.79,65.84 14.04,67.08 16.24,67.08 16.26,67.1 16.28,67.1 17.14,67.97 IC4.16
TIMBRE_POT
  Top 0.254: IC4.13 15.64,68.85 15.54,68.74 13.86,68.74 10.14,65.02 R7.P$2 10.14,53.12 C32.1
TX
  Top 0.203: 5.57,52.9 5.5,52.96 5.31,52.96 R10.2
  Top 0.254: 5.57,52.9 6.17,53.5 6.17,57.78 7.76,59.37 7.76,63.34 13.79,69.37 14.51,69.37 15.78,70.64 16.97,70.64 18.24,71.91 | 18.24,71.91 | 18.24,71.91 18.24,75.72 17.14,76.81 IC4.45 | 18.24,71.91
V_OCT_IN
  Top 0.254: J8.P3 29.56,1.85 C60.1 36.12,1.85 38.08,3.81 38.08,13.02 39.35,14.29 39.35,17.14 39.98,17.78 41.57,17.78 42.21,17.14 50.14,17.14 51.41,18.41 52.68,18.41 54.27,20 54.27,31.43 53.64,32.07 51.41,32.07 48.24,35.24 48.24,37.47 46.02,39.69 28.55,39.69 27.6,38.73 27.6,35.36 26.97,34.72 22.88,34.72 22.34,35.26 R38.2
VCC
  Top 0.254: 43.48,96.52 C4.+ | IC8.8 52.41,46.67 51.41,46.67 51.41,48.26 C37.1
  Top 0.406: 43.48,96.52 43.48,93.98 45.7,91.76 53,91.76 55.54,89.22 55.54,53.02 51.83,49.31 C37.1 | L2.1 40.73,96.2 41.57,96.2 41.89,96.52 C4.+
VEE  (via drill 0.5)
  Top 0.254: C45.2 45.72,44.74 IC8.4 45.96,44.12 R37.1 46.53,42.86 v48.26,42.86
  Top 0.406: v55.22,48.58 55.22,51.75 56.18,52.7 56.18,89.53 53,92.71 53.01,92.72 C5.- 54.27,96.52 54.85,95.94 L3.1
  Bottom 0.406: v55.22,48.58 49.51,42.86 v48.26,42.86

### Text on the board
bNames: solder IC1 to this side, check polarity, email adam if unsure | +12V | GND | GND | GND | -12V | Red Stripe | Pilates0603 | cc-by-sa émilie gillet 2017 v5
tStop: cc-by-sa | 2017. v5 | émilie gillet | Pirate603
